(* Logix 5000 Program export BasicLaserCommands; software revision 21.03 *)

TYPE GENERIC :
STRUCT
   cmd : GENERIC_CMD;
   res : LSTRING;
   error : DINT;
END_STRUCT
END_TYPE

TYPE SIMPLECMD :
STRUCT
   cmd : EMPTY_CMD;
   res : LSTRING;
   error : DINT;
END_STRUCT
END_TYPE

TYPE GETCOUNT :
STRUCT
   cmd : GETID_CMD;
   res : DINT;
   error : DINT;
END_STRUCT
END_TYPE

TYPE GETVARIABLES :
STRUCT
   cmd : GETID_CMD;
   res : LSTRING;
   error : DINT;
END_STRUCT
END_TYPE

TYPE SETPOSITIONOFFSET :
STRUCT
   cmd : SETPOSITIONOFFSET_CMD;
   error : DINT;
END_STRUCT
END_TYPE

TYPE SETDATA :
STRUCT
   cmd : SETDATA_CMD;
   error : DINT;
END_STRUCT
END_TYPE

TYPE LSTRING :   // string type
STRUCT
   LEN : DINT;
   DATA : SINT[400];
END_STRUCT
END_TYPE

TYPE SETENCODERDELAY_CMD :
STRUCT
   value : LSTRING;
   global : BOOL;
   send : BOOL;
END_STRUCT
END_TYPE

TYPE GETCOUNTERVALUE :
STRUCT
   cmd : GETID_CMD;
   res : LSTRING;
   error : DINT;
END_STRUCT
END_TYPE

TYPE BasicLaserCommands :
STRUCT
   BEGINTRANS : NORES_CMD;
   EXECTRANS : NORES_CMD;
   GETCOUNT : GETCOUNT;
   SETCOUNT : SETCOUNT;
   GETCOUNTERVALUE : GETCOUNTERVALUE;
   SETCOUNTERVALUE : SETCOUNTERVALUE;
   GETPARSEDTEXT : GETPARSEDTEXT;
   GETTEXT : GETTEXT;
   SETTEXT : SETTEXT;
   GETVARLIST : SIMPLECMD;
   GETVARIABLES : GETVARIABLES;
   SETVARIABLES : SETVARIABLES;
   LOADPROJECT : LOADPROJECT;
   GETCURRENTPROJECT : SIMPLECMD;
   SAVEPROJECT : SAVEPROJECT;
   GETPOSITIONOFFSET : GETPOSITIONOFFSET;
   SETPOSITIONOFFSET : SETPOSITIONOFFSET;
   GETENCODERDELAY : GETENCODERDELAY;
   SETENCODERDELAY : SETENCODERDELAY;
   RESETSYSTEM : NORES_CMD;
   GETDATA : GETDATA;
   SETDATA : SETDATA;
   GETVERSION : GETVERSION;
   GENERIC : GENERIC;
   priv : LASER_PRIVATE_FIELDS;
END_STRUCT
END_TYPE

TYPE SAVEPROJECT :
STRUCT
   cmd : LOADPROJECT_CMD;
   error : DINT;
END_STRUCT
END_TYPE

TYPE LASER_PRIVATE_FIELDS :
STRUCT
   data : SINT[808];
   busy : BOOL;
END_STRUCT
END_TYPE

TYPE GETDATA_CMD :
STRUCT
   object : LSTRING;
   id : LSTRING;
   send : BOOL;
END_STRUCT
END_TYPE

TYPE GETENCODERDELAY :
STRUCT
   cmd : GETENCODERDELAY_CMD;
   res : LSTRING;
   error : DINT;
END_STRUCT
END_TYPE

TYPE SETCOUNT :
STRUCT
   cmd : SETCOUNT_CMD;
   error : DINT;
END_STRUCT
END_TYPE

TYPE GETID_CMD :
STRUCT
   ID : LSTRING;
   send : BOOL;
END_STRUCT
END_TYPE

TYPE POSITION :
STRUCT
   x : REAL;
   y : REAL;
END_STRUCT
END_TYPE

TYPE GETENCODERDELAY_CMD :
STRUCT
   global : BOOL;
   send : BOOL;
END_STRUCT
END_TYPE

TYPE SETDATA_CMD :
STRUCT
   object : LSTRING;
   id : LSTRING;
   data : LSTRING;
   send : BOOL;
END_STRUCT
END_TYPE

TYPE SETVARIABLES :
STRUCT
   cmd : SETID_CMD;
   error : DINT;
END_STRUCT
END_TYPE

TYPE GETDATA :
STRUCT
   cmd : GETDATA_CMD;
   res : LSTRING;
   error : DINT;
END_STRUCT
END_TYPE

TYPE GETPOSITIONOFFSET :
STRUCT
   cmd : EMPTY_CMD;
   res : POSITION;
   error : DINT;
END_STRUCT
END_TYPE

TYPE SETCOUNTERVALUE :
STRUCT
   cmd : SETID_CMD;
   error : DINT;
END_STRUCT
END_TYPE

TYPE SETPOSITIONOFFSET_CMD :
STRUCT
   pos : POSITION;
   send : BOOL;
END_STRUCT
END_TYPE

TYPE EMPTY_CMD :
STRUCT
   send : BOOL;
END_STRUCT
END_TYPE

TYPE SETENCODERDELAY :
STRUCT
   cmd : SETENCODERDELAY_CMD;
   error : DINT;
END_STRUCT
END_TYPE

TYPE SETID_CMD :
STRUCT
   ID : LSTRING;
   value : LSTRING;
   send : BOOL;
END_STRUCT
END_TYPE

TYPE LOADPROJECT :
STRUCT
   cmd : LOADPROJECT_CMD;
   error : DINT;
END_STRUCT
END_TYPE

TYPE LOADPROJECT_CMD :
STRUCT
   URI : LSTRING;
   send : BOOL;
END_STRUCT
END_TYPE

TYPE GETVERSION :
STRUCT
   cmd : EMPTY_CMD;
   res : GETVERSION_RES;
   error : DINT;
END_STRUCT
END_TYPE

TYPE SETTEXT_CMD :
STRUCT
   name : LSTRING;
   value : LSTRING;
   send : BOOL;
END_STRUCT
END_TYPE

TYPE GETVERSION_RES :
STRUCT
   software : LSTRING;
   dsp : LSTRING;
   image : LSTRING;
END_STRUCT
END_TYPE

TYPE GENERIC_CMD :
STRUCT
   command : LSTRING;
   arg2 : LSTRING;
   arg3 : LSTRING;
   arg4 : LSTRING;
   arg5 : LSTRING;
   send : BOOL;
END_STRUCT
END_TYPE

TYPE GETTEXT_CMD :
STRUCT
   name : LSTRING;
   send : BOOL;
END_STRUCT
END_TYPE

TYPE GETPARSEDTEXT :
STRUCT
   cmd : GETTEXT_CMD;
   res : LSTRING;
   error : DINT;
END_STRUCT
END_TYPE

TYPE SETTEXT :
STRUCT
   cmd : SETTEXT_CMD;
   error : DINT;
END_STRUCT
END_TYPE

TYPE SETCOUNT_CMD :
STRUCT
   ID : LSTRING;
   value : DINT;
   send : BOOL;
END_STRUCT
END_TYPE

TYPE NORES_CMD :
STRUCT
   cmd : EMPTY_CMD;
   error : DINT;
END_STRUCT
END_TYPE

TYPE GETTEXT :
STRUCT
   cmd : GETTEXT_CMD;
   res : LSTRING;
   error : DINT;
END_STRUCT
END_TYPE

ADD_ON_INSTRUCTION StrToArr   (* revision 1.0, vendor 1 *)
VAR_IN_OUT
   out : SINT[404]; {required}
   str : LSTRING; {required}
END_VAR
VAR_OUTPUT
   size : DINT; {access Read Only, required}
END_VAR

ROUTINE Logic   (* ladder *)
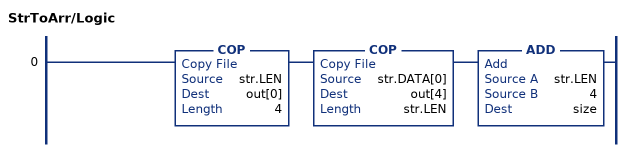
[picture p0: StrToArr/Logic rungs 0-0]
   0: COP(str.LEN,out[0],4)COP(str.DATA[0],out[4],str.LEN)ADD(str.LEN,4,size);
END_ROUTINE
END_ADD_ON_INSTRUCTION

ADD_ON_INSTRUCTION AppendStrs   (* revision 1.0, vendor 1 *)
VAR_IN_OUT
   str1 : LSTRING; {required}
   str2 : LSTRING; {required}
   out : SINT[808]; {required}
END_VAR
VAR_OUTPUT
   size : DINT; {access Read Only, required}
END_VAR
VAR
   cpy : StrToArr; {access None}
   n : DINT; {access None}
   offset : DINT; {access None}
   buf : SINT[404]; {access None}
END_VAR

ROUTINE Logic   (* ladder *)
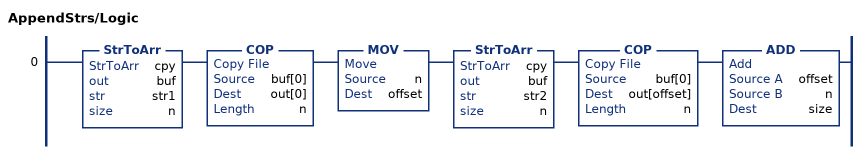
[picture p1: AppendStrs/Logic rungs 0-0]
   0: StrToArr(cpy,buf,str1,n)COP(buf[0],out[0],n)MOV(n,offset)StrToArr(cpy,buf,str2,n)COP(buf[0],out[offset],n)ADD(offset,n,size);
END_ROUTINE
END_ADD_ON_INSTRUCTION

ADD_ON_INSTRUCTION AppendStrs5   (* revision 1.0, vendor 1 *)
VAR_IN_OUT
   str1 : LSTRING; {required}
   str2 : LSTRING; {required}
   str3 : LSTRING; {required}
   str4 : LSTRING; {required}
   str5 : LSTRING; {required}
   out : SINT[808]; {required}
END_VAR
VAR_OUTPUT
   size : DINT; {access Read Only, required}
END_VAR
VAR_INPUT
   number_of_strings : DINT; {required}
   offset : DINT; {required}
END_VAR
VAR
   cpy : StrToArr; {access None}
   n : DINT; {access None}
   buf : SINT[404]; {access None}
END_VAR

ROUTINE Logic   (* ladder *)
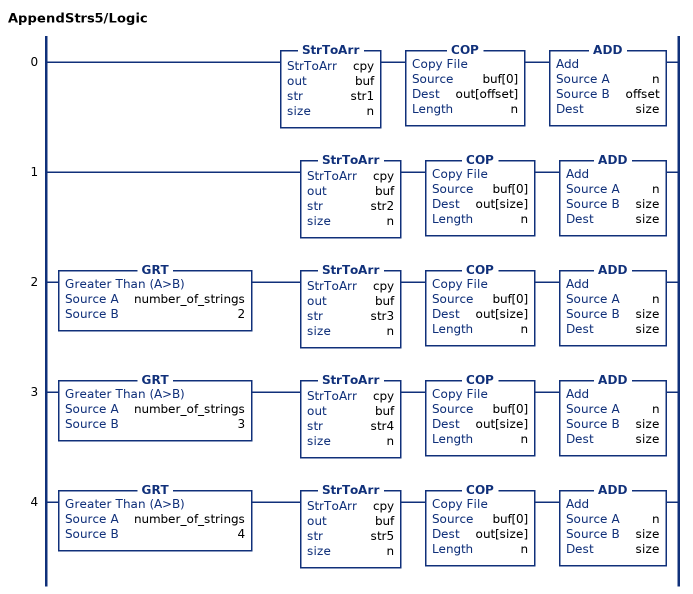
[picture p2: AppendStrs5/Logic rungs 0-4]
   0: StrToArr(cpy,buf,str1,n)COP(buf[0],out[offset],n)ADD(n,offset,size);
   1: StrToArr(cpy,buf,str2,n)COP(buf[0],out[size],n)ADD(n,size,size);
   2: GRT(number_of_strings,2)StrToArr(cpy,buf,str3,n)COP(buf[0],out[size],n)ADD(n,size,size);
   3: GRT(number_of_strings,3)StrToArr(cpy,buf,str4,n)COP(buf[0],out[size],n)ADD(n,size,size);
   4: GRT(number_of_strings,4)StrToArr(cpy,buf,str5,n)COP(buf[0],out[size],n)ADD(n,size,size);
END_ROUTINE
END_ADD_ON_INSTRUCTION

ADD_ON_INSTRUCTION ArrToStr   (* revision 1.0, vendor 1 *)
VAR_IN_OUT
   arr : SINT[404]; {required}
   out : LSTRING; {required}
END_VAR

ROUTINE Logic   (* ladder *)
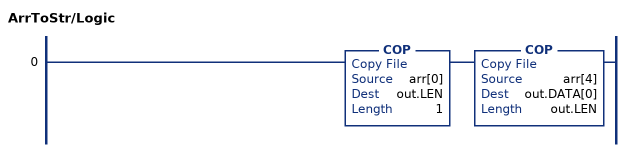
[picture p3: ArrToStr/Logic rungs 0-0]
   0: COP(arr[0],out.LEN,1)COP(arr[4],out.DATA[0],out.LEN);
END_ROUTINE
END_ADD_ON_INSTRUCTION

VAR_GLOBAL   (* controller tags *)
   Domino_internal_getvarlist : MESSAGE;
        MessageParameters(MessageType := CIP Generic, ConnectedFlag := 2, ConnectionPath := DFSeries, ServiceCode := 16#0054, ObjectType := 16#0064, TargetObject := 1, LocalElement := DFSeriesBasic.priv.data, DestinationTag := DFSeriesBasic.priv.data)
   Domino_internal_exectrans : MESSAGE;
        MessageParameters(MessageType := CIP Generic, ConnectedFlag := 2, ConnectionPath := DFSeries, ServiceCode := 16#004c, ObjectType := 16#0064, TargetObject := 1, LocalElement := DFSeriesBasic.priv, DestinationTag := DFSeriesBasic.priv)
   Domino_internal_gettext : MESSAGE;
        MessageParameters(MessageType := CIP Generic, RequestedLength := 101, ConnectedFlag := 2, ConnectionPath := DFSeries, ServiceCode := 16#0052, ObjectType := 16#0064, TargetObject := 1, LocalElement := DFSeriesBasic.priv, DestinationTag := DFSeriesBasic.priv)
   Domino_internal_loadproject : MESSAGE;
        MessageParameters(MessageType := CIP Generic, RequestedLength := 1, ConnectedFlag := 2, ConnectionPath := DFSeries, ServiceCode := 16#0057, ObjectType := 16#0064, TargetObject := 1, LocalElement := DFSeriesBasic.priv, DestinationTag := DFSeriesBasic.priv)
   Domino_internal_getcurrentproject : MESSAGE;
        MessageParameters(MessageType := CIP Generic, ConnectedFlag := 2, ConnectionPath := DFSeries, ServiceCode := 16#0058, ObjectType := 16#0064, TargetObject := 1, LocalElement := DFSeriesBasic.priv, DestinationTag := DFSeriesBasic.priv)
   Domino_internal_getpositionoffset : MESSAGE;
        MessageParameters(MessageType := CIP Generic, ConnectedFlag := 2, ConnectionPath := DFSeries, ServiceCode := 16#005a, ObjectType := 16#0064, TargetObject := 1, LocalElement := DFSeriesBasic.priv, DestinationTag := DFSeriesBasic.priv)
   Domino_internal_setcountervalue : MESSAGE;
        MessageParameters(MessageType := CIP Generic, RequestedLength := 1, ConnectedFlag := 2, ConnectionPath := DFSeries, ServiceCode := 16#0050, ObjectType := 16#0064, TargetObject := 1, LocalElement := DFSeriesBasic.priv, DestinationTag := DFSeriesBasic.priv)
   Domino_internal_setcount : MESSAGE;
        MessageParameters(MessageType := CIP Generic, RequestedLength := 1, ConnectedFlag := 2, ConnectionPath := DFSeries, ServiceCode := 16#004e, ObjectType := 16#0064, TargetObject := 1, LocalElement := DFSeriesBasic.priv, DestinationTag := DFSeriesBasic.priv)
   DFSeriesBasic : BasicLaserCommands;
   Domino_internal_resetsystem : MESSAGE;
        MessageParameters(MessageType := CIP Generic, ConnectedFlag := 2, ConnectionPath := DFSeries, ServiceCode := 16#005e, ObjectType := 16#0064, TargetObject := 1, LocalElement := DFSeriesBasic.priv, DestinationTag := DFSeriesBasic.priv)
   Domino_internal_getdata : MESSAGE;
        MessageParameters(MessageType := CIP Generic, RequestedLength := 1, ConnectedFlag := 2, ConnectionPath := DFSeries, ServiceCode := 16#005f, ObjectType := 16#0064, TargetObject := 1, LocalElement := DFSeriesBasic.priv, DestinationTag := DFSeriesBasic.priv)
   Domino_internal_getencoderdelay : MESSAGE;
        MessageParameters(MessageType := CIP Generic, RequestedLength := 1, ConnectedFlag := 2, ConnectionPath := DFSeries, ServiceCode := 16#005c, ObjectType := 16#0064, TargetObject := 1, LocalElement := DFSeriesBasic.priv, DestinationTag := DFSeriesBasic.priv)
   Domino_internal_generic : MESSAGE;
        MessageParameters(MessageType := CIP Generic, RequestedLength := 1, ConnectedFlag := 2, ConnectionPath := DFSeries, ServiceCode := 16#0063, ObjectType := 16#0064, TargetObject := 1, LocalElement := DFSeriesBasic.priv, DestinationTag := DFSeriesBasic.priv)
   Domino_internal_setvariables : MESSAGE;
        MessageParameters(MessageType := CIP Generic, RequestedLength := 1, ConnectedFlag := 2, ConnectionPath := DFSeries, ServiceCode := 16#0056, ObjectType := 16#0064, TargetObject := 1, LocalElement := DFSeriesBasic.priv, DestinationTag := DFSeriesBasic.priv)
   Domino_internal_getcountervalue : MESSAGE;
        MessageParameters(MessageType := CIP Generic, RequestedLength := 1, ConnectedFlag := 2, ConnectionPath := DFSeries, ServiceCode := 16#004f, ObjectType := 16#0064, TargetObject := 1, LocalElement := DFSeriesBasic.priv, DestinationTag := DFSeriesBasic.priv)
   Domino_internal_setpositionoffset : MESSAGE;
        MessageParameters(MessageType := CIP Generic, RequestedLength := 8, ConnectedFlag := 2, ConnectionPath := DFSeries, ServiceCode := 16#005b, ObjectType := 16#0064, TargetObject := 1, LocalElement := DFSeriesBasic.priv, DestinationTag := DFSeriesBasic.priv)
   Domino_internal_setencoderdelay : MESSAGE;
        MessageParameters(MessageType := CIP Generic, RequestedLength := 1, ConnectedFlag := 2, ConnectionPath := DFSeries, ServiceCode := 16#005d, ObjectType := 16#0064, TargetObject := 1, LocalElement := DFSeriesBasic.priv, DestinationTag := DFSeriesBasic.priv)
   Domino_internal_setdata : MESSAGE;
        MessageParameters(MessageType := CIP Generic, RequestedLength := 1, ConnectedFlag := 2, ConnectionPath := DFSeries, ServiceCode := 16#0060, ObjectType := 16#0064, TargetObject := 1, LocalElement := DFSeriesBasic.priv, DestinationTag := DFSeriesBasic.priv)
   Domino_internal_getparsedtext : MESSAGE;
        MessageParameters(MessageType := CIP Generic, RequestedLength := 1, ConnectedFlag := 2, ConnectionPath := DFSeries, ServiceCode := 16#0051, ObjectType := 16#0064, TargetObject := 1, LocalElement := DFSeriesBasic.priv, DestinationTag := DFSeriesBasic.priv)
   Domino_internal_getversion : MESSAGE;
        MessageParameters(MessageType := CIP Generic, ConnectedFlag := 2, ConnectionPath := DFSeries, ServiceCode := 16#0061, ObjectType := 16#0064, TargetObject := 1, LocalElement := DFSeriesBasic.priv, DestinationTag := DFSeriesBasic.priv)
   Domino_internal_begintrans : MESSAGE;
        MessageParameters(MessageType := CIP Generic, ConnectedFlag := 2, ConnectionPath := DFSeries, ServiceCode := 16#004b, ObjectType := 16#0064, TargetObject := 1, LocalElement := DFSeriesBasic.priv, DestinationTag := DFSeriesBasic.priv)
   Domino_internal_getvariables : MESSAGE;
        MessageParameters(MessageType := CIP Generic, RequestedLength := 1, ConnectedFlag := 2, ConnectionPath := DFSeries, ServiceCode := 16#0055, ObjectType := 16#0064, TargetObject := 1, LocalElement := DFSeriesBasic.priv, DestinationTag := DFSeriesBasic.priv)
   Domino_internal_settext : MESSAGE;
        MessageParameters(MessageType := CIP Generic, RequestedLength := 202, ConnectedFlag := 2, ConnectionPath := DFSeries, ServiceCode := 16#0053, ObjectType := 16#0064, TargetObject := 1, LocalElement := DFSeriesBasic.priv, DestinationTag := DFSeriesBasic.priv)
   Domino_internal_saveproject : MESSAGE;
        MessageParameters(MessageType := CIP Generic, RequestedLength := 1, ConnectedFlag := 2, ConnectionPath := DFSeries, ServiceCode := 16#0059, ObjectType := 16#0064, TargetObject := 1, LocalElement := DFSeriesBasic.priv, DestinationTag := DFSeriesBasic.priv)
   Domino_internal_getcount : MESSAGE;
        MessageParameters(MessageType := CIP Generic, RequestedLength := 1, ConnectedFlag := 2, ConnectionPath := DFSeries, ServiceCode := 16#004d, ObjectType := 16#0064, TargetObject := 1, LocalElement := DFSeriesBasic.priv, DestinationTag := DFSeriesBasic.priv)
END_VAR

PROGRAM BasicLaserCommands   (* main routine Main *)
VAR
   app : AppendStrs;
   app5 : AppendStrs5 := (number_of_strings := 3);
   len : DINT;
   n : DINT;
   toArr : StrToArr;
   toStr : ArrToStr;
END_VAR

ROUTINE Main   (* ladder *)
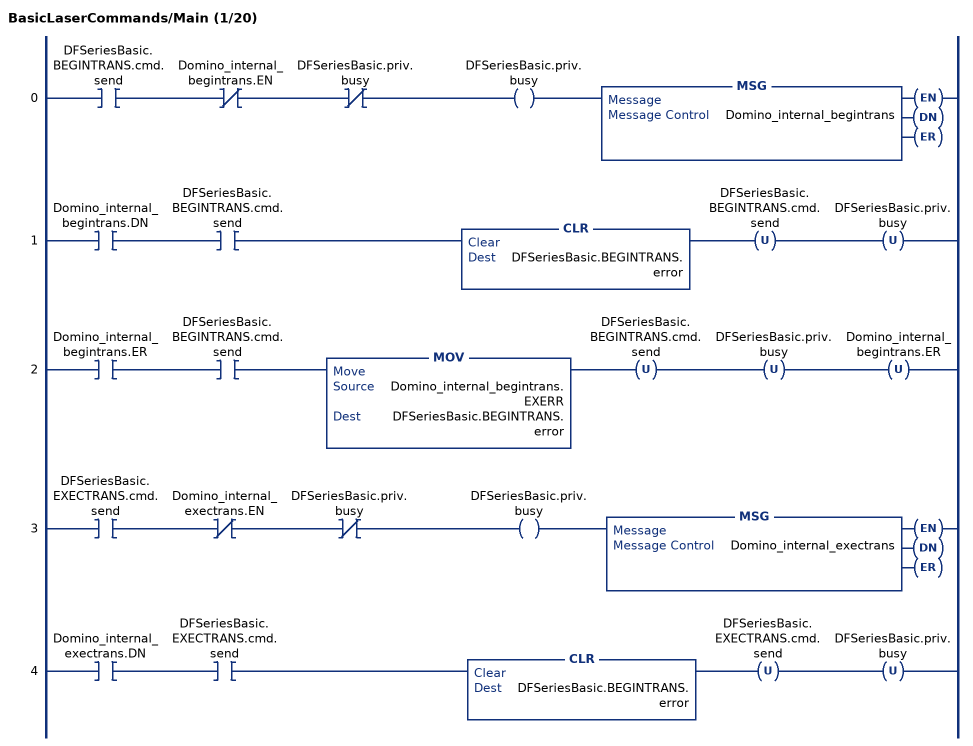
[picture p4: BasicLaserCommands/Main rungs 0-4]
   0: XIC(DFSeriesBasic.BEGINTRANS.cmd.send)XIO(Domino_internal_begintrans.EN)XIO(DFSeriesBasic.priv.busy)OTE(DFSeriesBasic.priv.busy)MSG(Domino_internal_begintrans);
   1: XIC(Domino_internal_begintrans.DN)XIC(DFSeriesBasic.BEGINTRANS.cmd.send)CLR(DFSeriesBasic.BEGINTRANS.error)OTU(DFSeriesBasic.BEGINTRANS.cmd.send)OTU(DFSeriesBasic.priv.busy);
   2: XIC(Domino_internal_begintrans.ER)XIC(DFSeriesBasic.BEGINTRANS.cmd.send)MOV(Domino_internal_begintrans.EXERR,DFSeriesBasic.BEGINTRANS.error)OTU(DFSeriesBasic.BEGINTRANS.cmd.send)OTU(DFSeriesBasic.priv.busy)OTU(Domino_internal_begintrans.ER);
   3: XIC(DFSeriesBasic.EXECTRANS.cmd.send)XIO(Domino_internal_exectrans.EN)XIO(DFSeriesBasic.priv.busy)OTE(DFSeriesBasic.priv.busy)MSG(Domino_internal_exectrans);
   4: XIC(Domino_internal_exectrans.DN)XIC(DFSeriesBasic.EXECTRANS.cmd.send)CLR(DFSeriesBasic.BEGINTRANS.error)OTU(DFSeriesBasic.EXECTRANS.cmd.send)OTU(DFSeriesBasic.priv.busy);
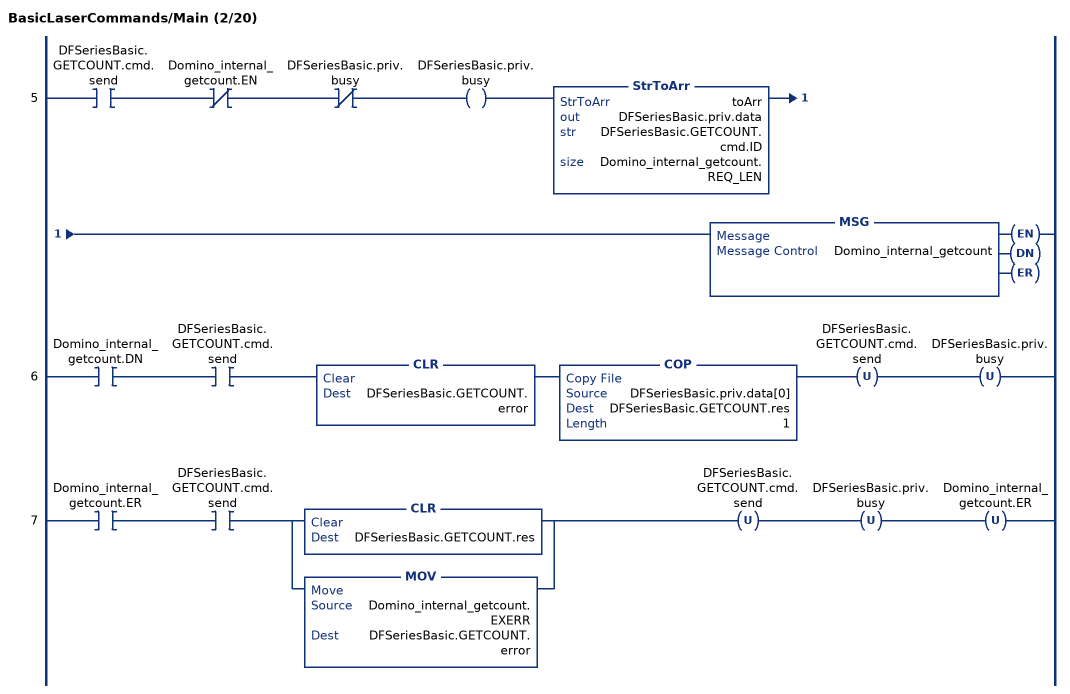
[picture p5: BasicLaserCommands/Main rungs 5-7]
   5: XIC(DFSeriesBasic.GETCOUNT.cmd.send)XIO(Domino_internal_getcount.EN)XIO(DFSeriesBasic.priv.busy)OTE(DFSeriesBasic.priv.busy)StrToArr(toArr,DFSeriesBasic.priv.data,DFSeriesBasic.GETCOUNT.cmd.ID,Domino_internal_getcount.REQ_LEN)MSG(Domino_internal_getcount);
   6: XIC(Domino_internal_getcount.DN)XIC(DFSeriesBasic.GETCOUNT.cmd.send)CLR(DFSeriesBasic.GETCOUNT.error)COP(DFSeriesBasic.priv.data[0],DFSeriesBasic.GETCOUNT.res,1)OTU(DFSeriesBasic.GETCOUNT.cmd.send)OTU(DFSeriesBasic.priv.busy);
   7: XIC(Domino_internal_getcount.ER)XIC(DFSeriesBasic.GETCOUNT.cmd.send)[CLR(DFSeriesBasic.GETCOUNT.res) ,MOV(Domino_internal_getcount.EXERR,DFSeriesBasic.GETCOUNT.error) ]OTU(DFSeriesBasic.GETCOUNT.cmd.send)OTU(DFSeriesBasic.priv.busy)OTU(Domino_internal_getcount.ER);
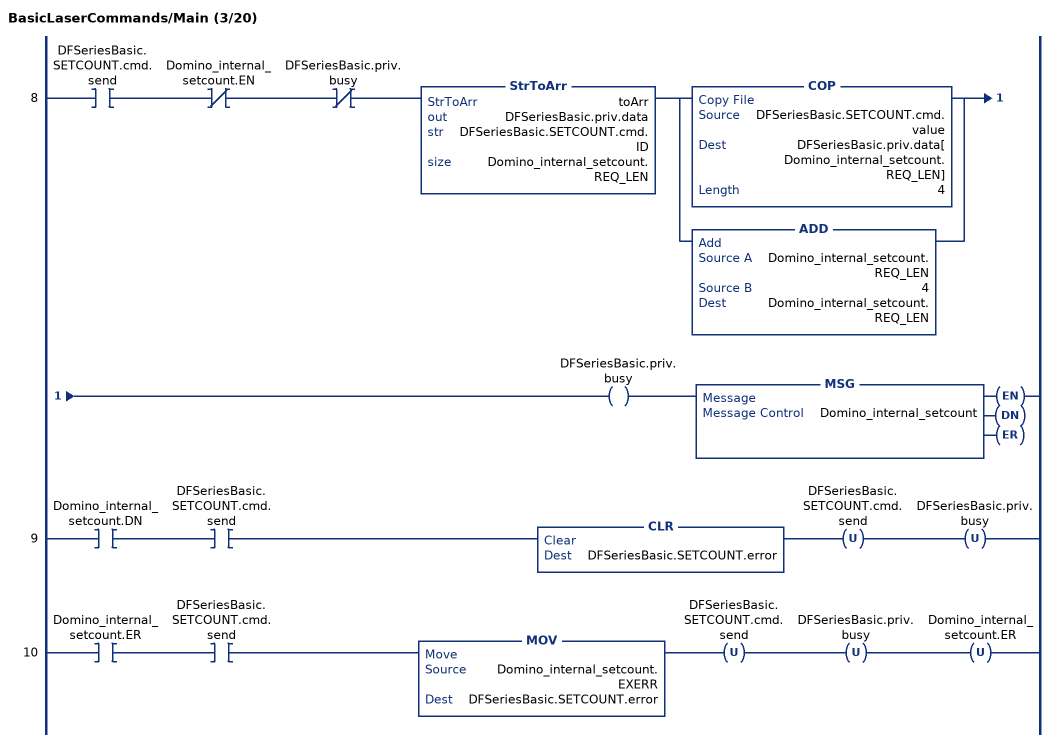
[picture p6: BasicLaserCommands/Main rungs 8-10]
   8: XIC(DFSeriesBasic.SETCOUNT.cmd.send)XIO(Domino_internal_setcount.EN)XIO(DFSeriesBasic.priv.busy)StrToArr(toArr,DFSeriesBasic.priv.data,DFSeriesBasic.SETCOUNT.cmd.ID,Domino_internal_setcount.REQ_LEN)[COP(DFSeriesBasic.SETCOUNT.cmd.value,DFSeriesBasic.priv.data[Domino_internal_setcount.REQ_LEN],4) ,ADD(Domino_internal_setcount.REQ_LEN,4,Domino_internal_setcount.REQ_LEN) ]OTE(DFSeriesBasic.priv.busy)MSG(Domino_internal_setcount);
   9: XIC(Domino_internal_setcount.DN)XIC(DFSeriesBasic.SETCOUNT.cmd.send)CLR(DFSeriesBasic.SETCOUNT.error)OTU(DFSeriesBasic.SETCOUNT.cmd.send)OTU(DFSeriesBasic.priv.busy);
   10: XIC(Domino_internal_setcount.ER)XIC(DFSeriesBasic.SETCOUNT.cmd.send)MOV(Domino_internal_setcount.EXERR,DFSeriesBasic.SETCOUNT.error)OTU(DFSeriesBasic.SETCOUNT.cmd.send)OTU(DFSeriesBasic.priv.busy)OTU(Domino_internal_setcount.ER);
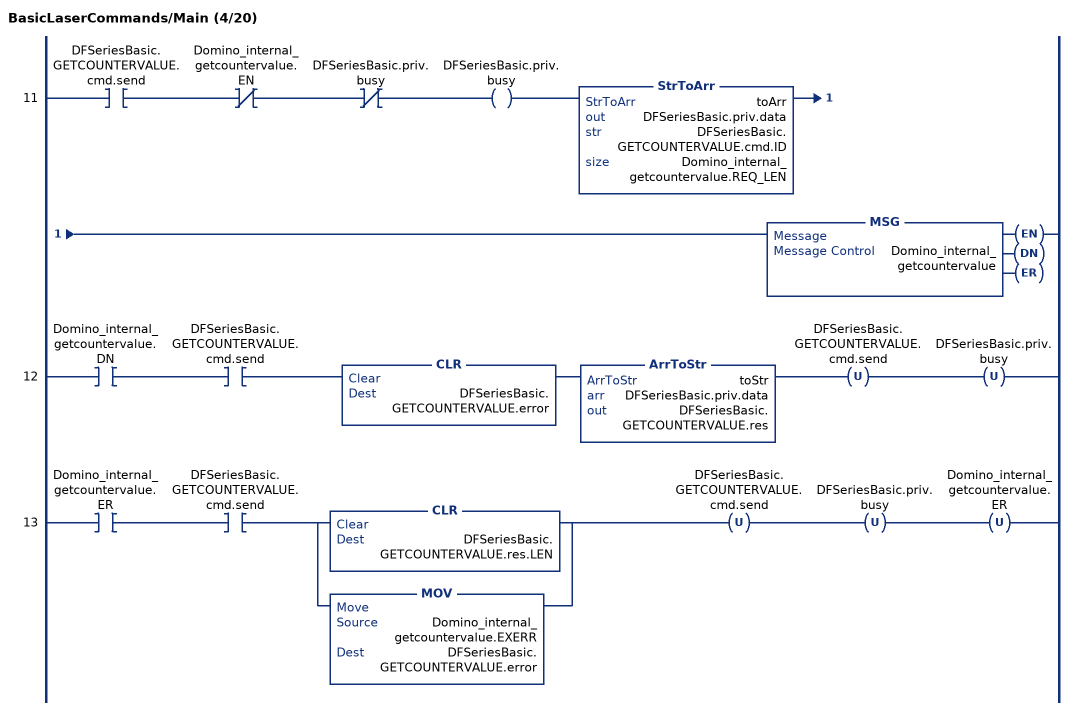
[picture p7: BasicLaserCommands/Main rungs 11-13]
   11: XIC(DFSeriesBasic.GETCOUNTERVALUE.cmd.send)XIO(Domino_internal_getcountervalue.EN)XIO(DFSeriesBasic.priv.busy)OTE(DFSeriesBasic.priv.busy)StrToArr(toArr,DFSeriesBasic.priv.data,DFSeriesBasic.GETCOUNTERVALUE.cmd.ID,Domino_internal_getcountervalue.REQ_LEN)MSG(Domino_internal_getcountervalue);
   12: XIC(Domino_internal_getcountervalue.DN)XIC(DFSeriesBasic.GETCOUNTERVALUE.cmd.send)CLR(DFSeriesBasic.GETCOUNTERVALUE.error)ArrToStr(toStr,DFSeriesBasic.priv.data,DFSeriesBasic.GETCOUNTERVALUE.res)OTU(DFSeriesBasic.GETCOUNTERVALUE.cmd.send)OTU(DFSeriesBasic.priv.busy);
   13: XIC(Domino_internal_getcountervalue.ER)XIC(DFSeriesBasic.GETCOUNTERVALUE.cmd.send)[CLR(DFSeriesBasic.GETCOUNTERVALUE.res.LEN) ,MOV(Domino_internal_getcountervalue.EXERR,DFSeriesBasic.GETCOUNTERVALUE.error) ]OTU(DFSeriesBasic.GETCOUNTERVALUE.cmd.send)OTU(DFSeriesBasic.priv.busy)OTU(Domino_internal_getcountervalue.ER);
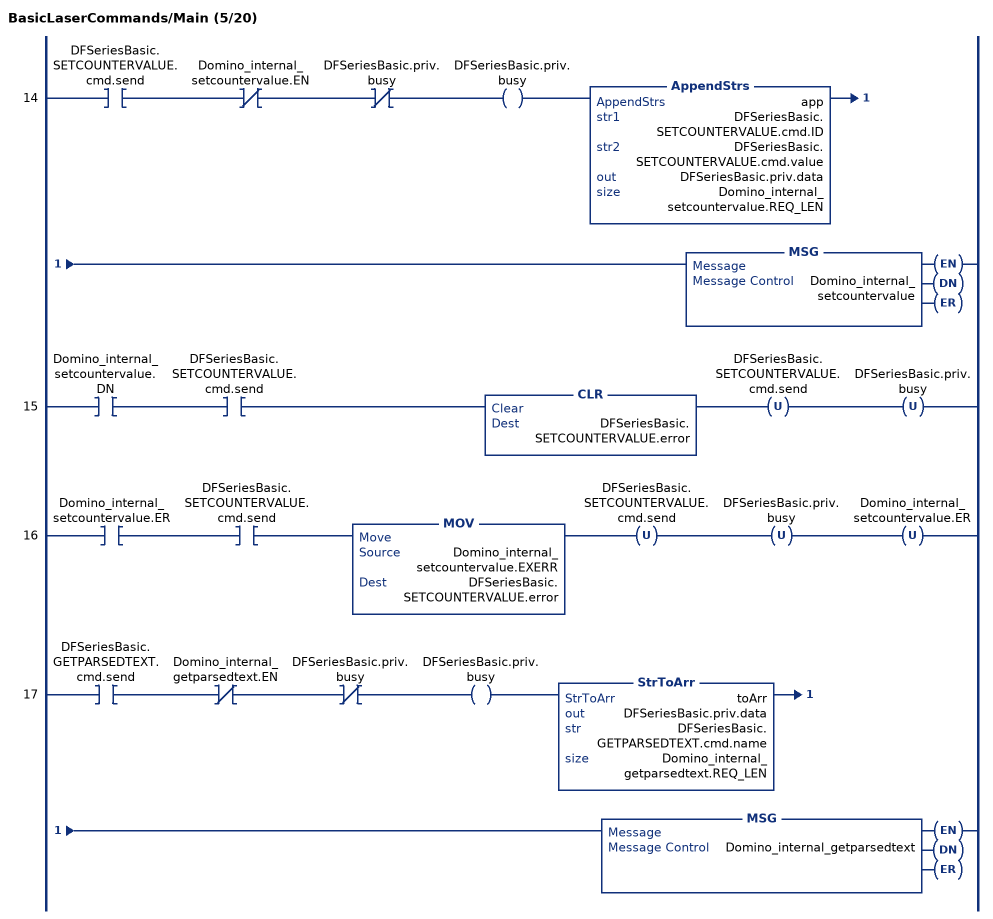
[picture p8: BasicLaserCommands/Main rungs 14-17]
   14: XIC(DFSeriesBasic.SETCOUNTERVALUE.cmd.send)XIO(Domino_internal_setcountervalue.EN)XIO(DFSeriesBasic.priv.busy)OTE(DFSeriesBasic.priv.busy)AppendStrs(app,DFSeriesBasic.SETCOUNTERVALUE.cmd.ID,DFSeriesBasic.SETCOUNTERVALUE.cmd.value,DFSeriesBasic.priv.data,Domino_internal_setcountervalue.REQ_LEN)MSG(Domino_internal_setcountervalue);
   15: XIC(Domino_internal_setcountervalue.DN)XIC(DFSeriesBasic.SETCOUNTERVALUE.cmd.send)CLR(DFSeriesBasic.SETCOUNTERVALUE.error)OTU(DFSeriesBasic.SETCOUNTERVALUE.cmd.send)OTU(DFSeriesBasic.priv.busy);
   16: XIC(Domino_internal_setcountervalue.ER)XIC(DFSeriesBasic.SETCOUNTERVALUE.cmd.send)MOV(Domino_internal_setcountervalue.EXERR,DFSeriesBasic.SETCOUNTERVALUE.error)OTU(DFSeriesBasic.SETCOUNTERVALUE.cmd.send)OTU(DFSeriesBasic.priv.busy)OTU(Domino_internal_setcountervalue.ER);
   17: XIC(DFSeriesBasic.GETPARSEDTEXT.cmd.send)XIO(Domino_internal_getparsedtext.EN)XIO(DFSeriesBasic.priv.busy)OTE(DFSeriesBasic.priv.busy)StrToArr(toArr,DFSeriesBasic.priv.data,DFSeriesBasic.GETPARSEDTEXT.cmd.name,Domino_internal_getparsedtext.REQ_LEN)MSG(Domino_internal_getparsedtext);
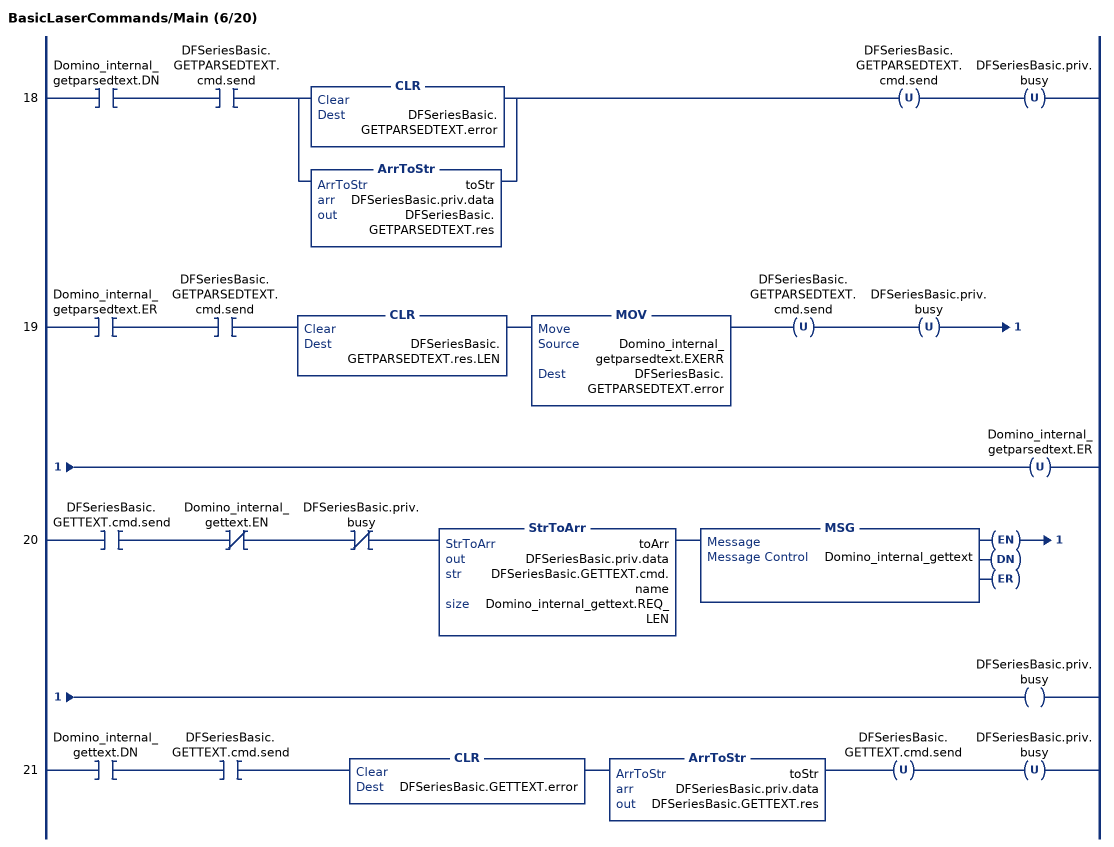
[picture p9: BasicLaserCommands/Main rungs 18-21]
   18: XIC(Domino_internal_getparsedtext.DN)XIC(DFSeriesBasic.GETPARSEDTEXT.cmd.send)[CLR(DFSeriesBasic.GETPARSEDTEXT.error) ,ArrToStr(toStr,DFSeriesBasic.priv.data,DFSeriesBasic.GETPARSEDTEXT.res) ]OTU(DFSeriesBasic.GETPARSEDTEXT.cmd.send)OTU(DFSeriesBasic.priv.busy);
   19: XIC(Domino_internal_getparsedtext.ER)XIC(DFSeriesBasic.GETPARSEDTEXT.cmd.send)CLR(DFSeriesBasic.GETPARSEDTEXT.res.LEN)MOV(Domino_internal_getparsedtext.EXERR,DFSeriesBasic.GETPARSEDTEXT.error)OTU(DFSeriesBasic.GETPARSEDTEXT.cmd.send)OTU(DFSeriesBasic.priv.busy)OTU(Domino_internal_getparsedtext.ER);
   20: XIC(DFSeriesBasic.GETTEXT.cmd.send)XIO(Domino_internal_gettext.EN)XIO(DFSeriesBasic.priv.busy)StrToArr(toArr,DFSeriesBasic.priv.data,DFSeriesBasic.GETTEXT.cmd.name,Domino_internal_gettext.REQ_LEN)MSG(Domino_internal_gettext)OTE(DFSeriesBasic.priv.busy);
   21: XIC(Domino_internal_gettext.DN)XIC(DFSeriesBasic.GETTEXT.cmd.send)CLR(DFSeriesBasic.GETTEXT.error)ArrToStr(toStr,DFSeriesBasic.priv.data,DFSeriesBasic.GETTEXT.res)OTU(DFSeriesBasic.GETTEXT.cmd.send)OTU(DFSeriesBasic.priv.busy);
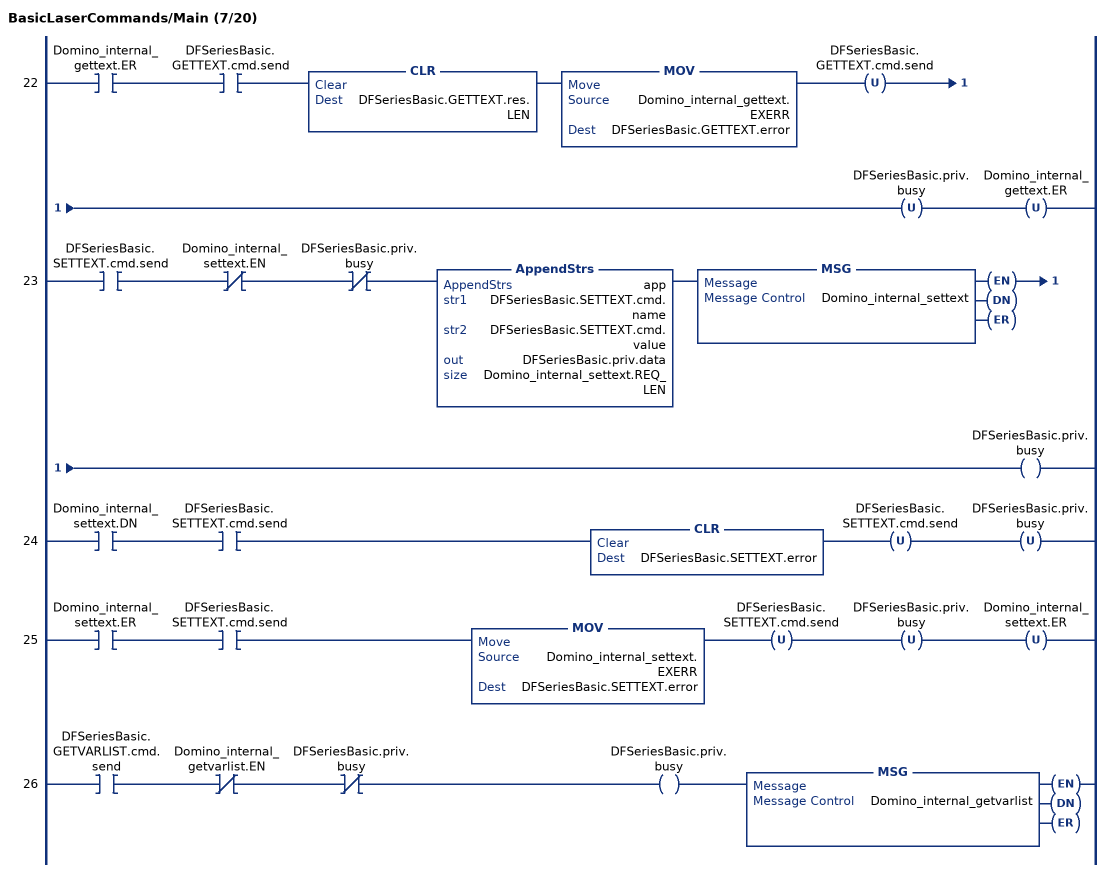
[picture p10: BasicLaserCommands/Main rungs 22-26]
   22: XIC(Domino_internal_gettext.ER)XIC(DFSeriesBasic.GETTEXT.cmd.send)CLR(DFSeriesBasic.GETTEXT.res.LEN)MOV(Domino_internal_gettext.EXERR,DFSeriesBasic.GETTEXT.error)OTU(DFSeriesBasic.GETTEXT.cmd.send)OTU(DFSeriesBasic.priv.busy)OTU(Domino_internal_gettext.ER);
   23: XIC(DFSeriesBasic.SETTEXT.cmd.send)XIO(Domino_internal_settext.EN)XIO(DFSeriesBasic.priv.busy)AppendStrs(app,DFSeriesBasic.SETTEXT.cmd.name,DFSeriesBasic.SETTEXT.cmd.value,DFSeriesBasic.priv.data,Domino_internal_settext.REQ_LEN)MSG(Domino_internal_settext)OTE(DFSeriesBasic.priv.busy);
   24: XIC(Domino_internal_settext.DN)XIC(DFSeriesBasic.SETTEXT.cmd.send)CLR(DFSeriesBasic.SETTEXT.error)OTU(DFSeriesBasic.SETTEXT.cmd.send)OTU(DFSeriesBasic.priv.busy);
   25: XIC(Domino_internal_settext.ER)XIC(DFSeriesBasic.SETTEXT.cmd.send)MOV(Domino_internal_settext.EXERR,DFSeriesBasic.SETTEXT.error)OTU(DFSeriesBasic.SETTEXT.cmd.send)OTU(DFSeriesBasic.priv.busy)OTU(Domino_internal_settext.ER);
   26: XIC(DFSeriesBasic.GETVARLIST.cmd.send)XIO(Domino_internal_getvarlist.EN)XIO(DFSeriesBasic.priv.busy)OTE(DFSeriesBasic.priv.busy)MSG(Domino_internal_getvarlist);
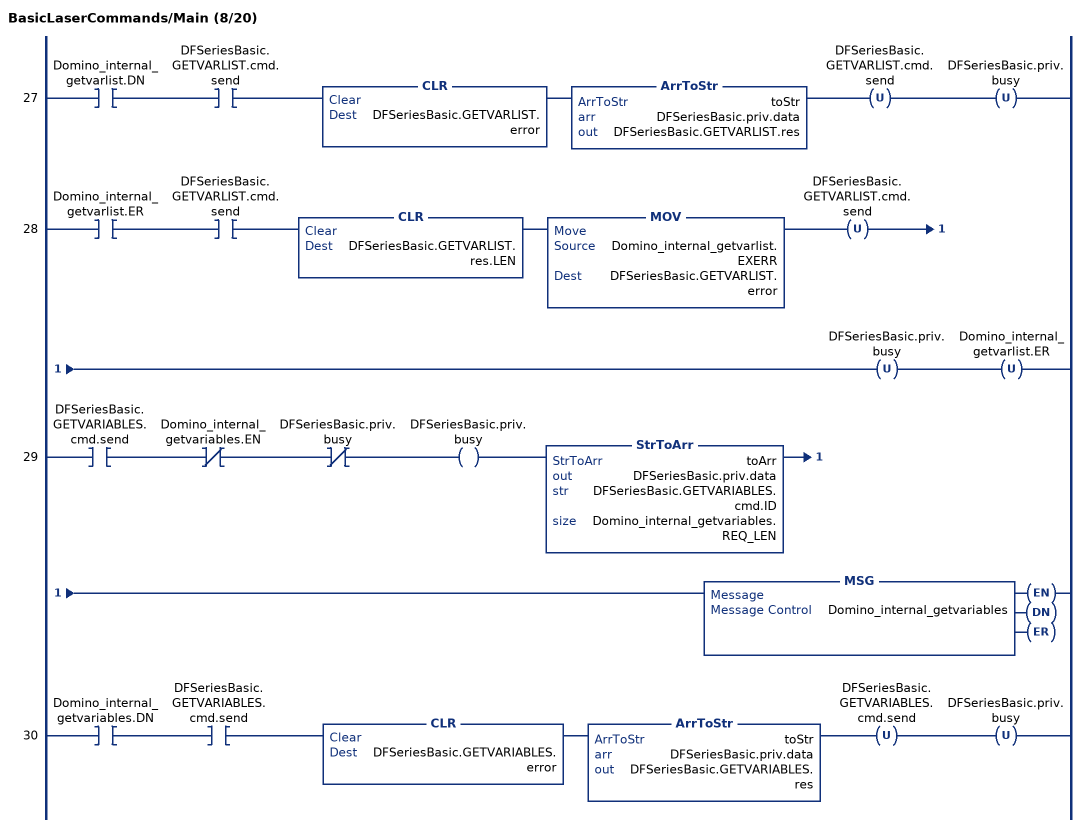
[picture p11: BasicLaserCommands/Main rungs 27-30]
   27: XIC(Domino_internal_getvarlist.DN)XIC(DFSeriesBasic.GETVARLIST.cmd.send)CLR(DFSeriesBasic.GETVARLIST.error)ArrToStr(toStr,DFSeriesBasic.priv.data,DFSeriesBasic.GETVARLIST.res)OTU(DFSeriesBasic.GETVARLIST.cmd.send)OTU(DFSeriesBasic.priv.busy);
   28: XIC(Domino_internal_getvarlist.ER)XIC(DFSeriesBasic.GETVARLIST.cmd.send)CLR(DFSeriesBasic.GETVARLIST.res.LEN)MOV(Domino_internal_getvarlist.EXERR,DFSeriesBasic.GETVARLIST.error)OTU(DFSeriesBasic.GETVARLIST.cmd.send)OTU(DFSeriesBasic.priv.busy)OTU(Domino_internal_getvarlist.ER);
   29: XIC(DFSeriesBasic.GETVARIABLES.cmd.send)XIO(Domino_internal_getvariables.EN)XIO(DFSeriesBasic.priv.busy)OTE(DFSeriesBasic.priv.busy)StrToArr(toArr,DFSeriesBasic.priv.data,DFSeriesBasic.GETVARIABLES.cmd.ID,Domino_internal_getvariables.REQ_LEN)MSG(Domino_internal_getvariables);
   30: XIC(Domino_internal_getvariables.DN)XIC(DFSeriesBasic.GETVARIABLES.cmd.send)CLR(DFSeriesBasic.GETVARIABLES.error)ArrToStr(toStr,DFSeriesBasic.priv.data,DFSeriesBasic.GETVARIABLES.res)OTU(DFSeriesBasic.GETVARIABLES.cmd.send)OTU(DFSeriesBasic.priv.busy);
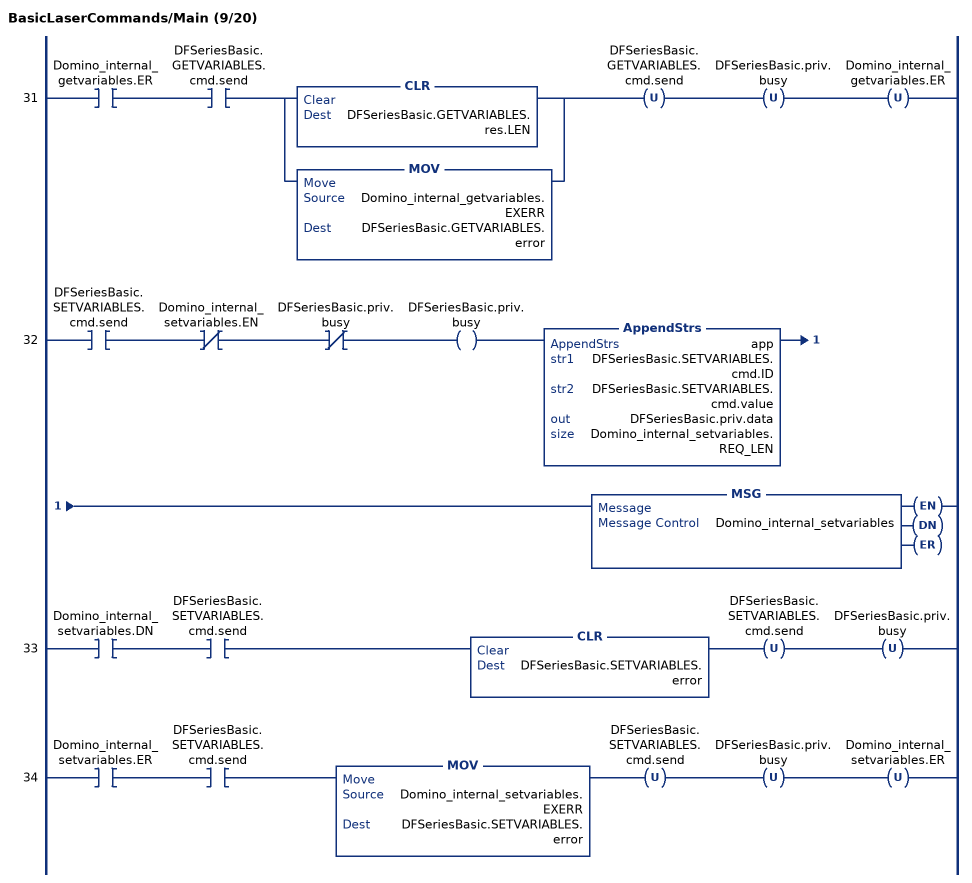
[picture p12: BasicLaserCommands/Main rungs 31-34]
   31: XIC(Domino_internal_getvariables.ER)XIC(DFSeriesBasic.GETVARIABLES.cmd.send)[CLR(DFSeriesBasic.GETVARIABLES.res.LEN) ,MOV(Domino_internal_getvariables.EXERR,DFSeriesBasic.GETVARIABLES.error) ]OTU(DFSeriesBasic.GETVARIABLES.cmd.send)OTU(DFSeriesBasic.priv.busy)OTU(Domino_internal_getvariables.ER);
   32: XIC(DFSeriesBasic.SETVARIABLES.cmd.send)XIO(Domino_internal_setvariables.EN)XIO(DFSeriesBasic.priv.busy)OTE(DFSeriesBasic.priv.busy)AppendStrs(app,DFSeriesBasic.SETVARIABLES.cmd.ID,DFSeriesBasic.SETVARIABLES.cmd.value,DFSeriesBasic.priv.data,Domino_internal_setvariables.REQ_LEN)MSG(Domino_internal_setvariables);
   33: XIC(Domino_internal_setvariables.DN)XIC(DFSeriesBasic.SETVARIABLES.cmd.send)CLR(DFSeriesBasic.SETVARIABLES.error)OTU(DFSeriesBasic.SETVARIABLES.cmd.send)OTU(DFSeriesBasic.priv.busy);
   34: XIC(Domino_internal_setvariables.ER)XIC(DFSeriesBasic.SETVARIABLES.cmd.send)MOV(Domino_internal_setvariables.EXERR,DFSeriesBasic.SETVARIABLES.error)OTU(DFSeriesBasic.SETVARIABLES.cmd.send)OTU(DFSeriesBasic.priv.busy)OTU(Domino_internal_setvariables.ER);
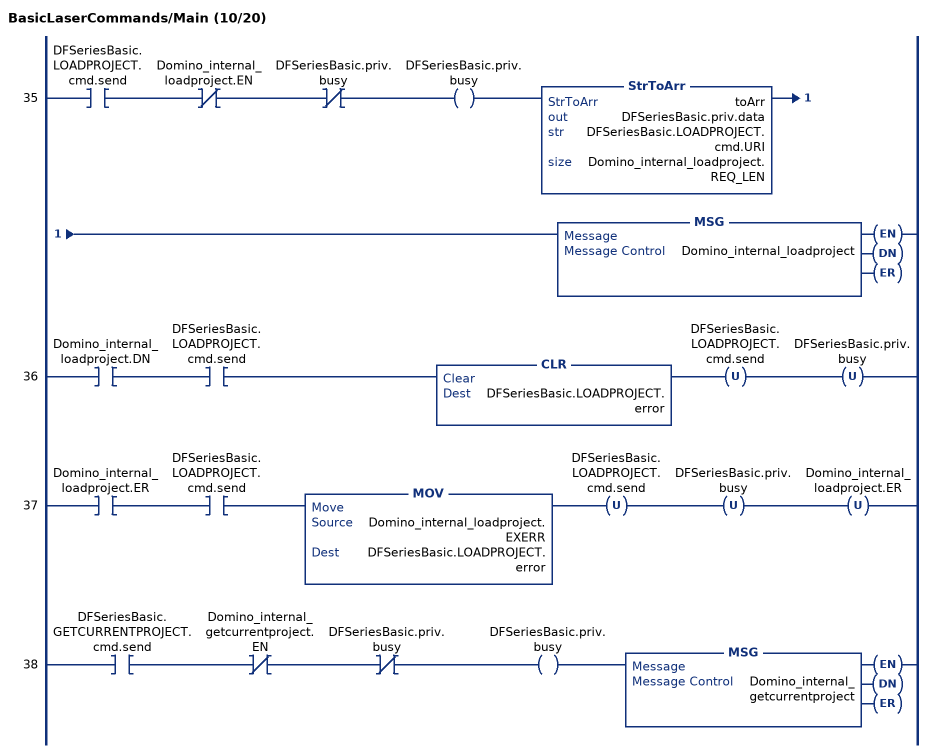
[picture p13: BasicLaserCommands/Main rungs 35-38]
   35: XIC(DFSeriesBasic.LOADPROJECT.cmd.send)XIO(Domino_internal_loadproject.EN)XIO(DFSeriesBasic.priv.busy)OTE(DFSeriesBasic.priv.busy)StrToArr(toArr,DFSeriesBasic.priv.data,DFSeriesBasic.LOADPROJECT.cmd.URI,Domino_internal_loadproject.REQ_LEN)MSG(Domino_internal_loadproject);
   36: XIC(Domino_internal_loadproject.DN)XIC(DFSeriesBasic.LOADPROJECT.cmd.send)CLR(DFSeriesBasic.LOADPROJECT.error)OTU(DFSeriesBasic.LOADPROJECT.cmd.send)OTU(DFSeriesBasic.priv.busy);
   37: XIC(Domino_internal_loadproject.ER)XIC(DFSeriesBasic.LOADPROJECT.cmd.send)MOV(Domino_internal_loadproject.EXERR,DFSeriesBasic.LOADPROJECT.error)OTU(DFSeriesBasic.LOADPROJECT.cmd.send)OTU(DFSeriesBasic.priv.busy)OTU(Domino_internal_loadproject.ER);
   38: XIC(DFSeriesBasic.GETCURRENTPROJECT.cmd.send)XIO(Domino_internal_getcurrentproject.EN)XIO(DFSeriesBasic.priv.busy)OTE(DFSeriesBasic.priv.busy)MSG(Domino_internal_getcurrentproject);
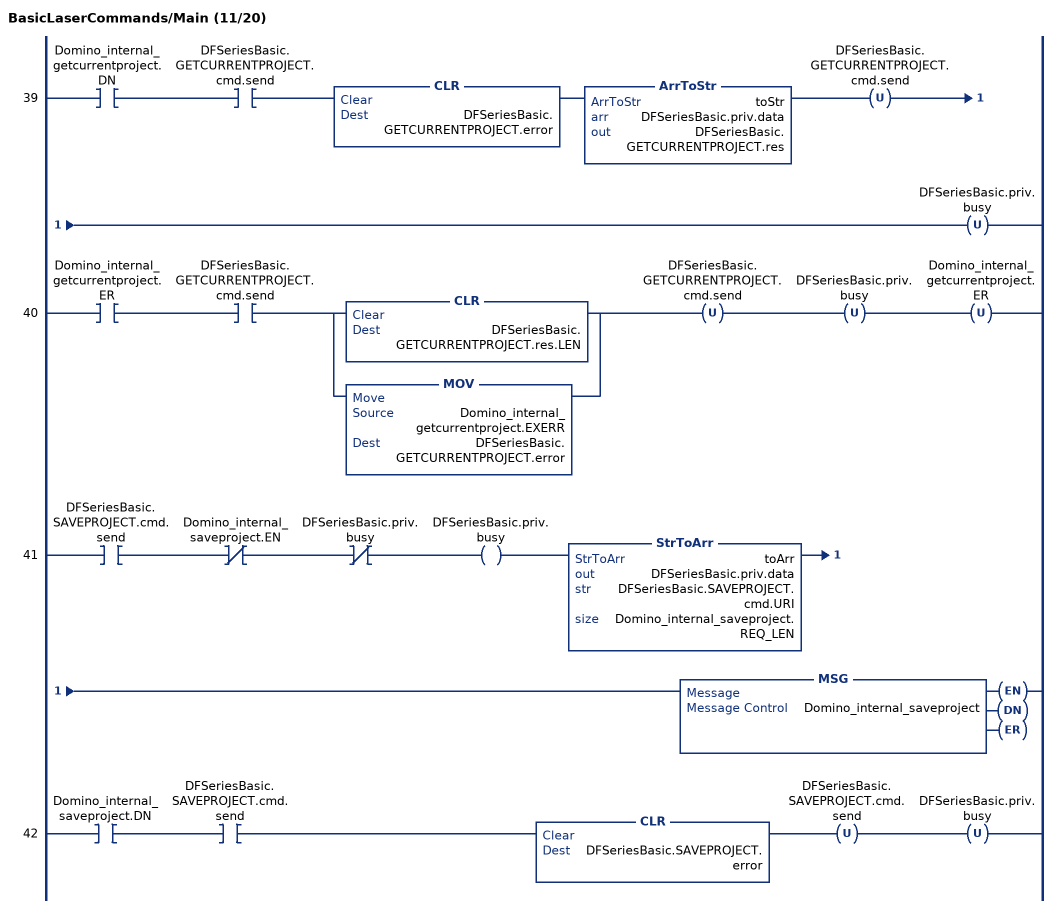
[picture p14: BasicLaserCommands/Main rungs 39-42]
   39: XIC(Domino_internal_getcurrentproject.DN)XIC(DFSeriesBasic.GETCURRENTPROJECT.cmd.send)CLR(DFSeriesBasic.GETCURRENTPROJECT.error)ArrToStr(toStr,DFSeriesBasic.priv.data,DFSeriesBasic.GETCURRENTPROJECT.res)OTU(DFSeriesBasic.GETCURRENTPROJECT.cmd.send)OTU(DFSeriesBasic.priv.busy);
   40: XIC(Domino_internal_getcurrentproject.ER)XIC(DFSeriesBasic.GETCURRENTPROJECT.cmd.send)[CLR(DFSeriesBasic.GETCURRENTPROJECT.res.LEN) ,MOV(Domino_internal_getcurrentproject.EXERR,DFSeriesBasic.GETCURRENTPROJECT.error) ]OTU(DFSeriesBasic.GETCURRENTPROJECT.cmd.send)OTU(DFSeriesBasic.priv.busy)OTU(Domino_internal_getcurrentproject.ER);
   41: XIC(DFSeriesBasic.SAVEPROJECT.cmd.send)XIO(Domino_internal_saveproject.EN)XIO(DFSeriesBasic.priv.busy)OTE(DFSeriesBasic.priv.busy)StrToArr(toArr,DFSeriesBasic.priv.data,DFSeriesBasic.SAVEPROJECT.cmd.URI,Domino_internal_saveproject.REQ_LEN)MSG(Domino_internal_saveproject);
   42: XIC(Domino_internal_saveproject.DN)XIC(DFSeriesBasic.SAVEPROJECT.cmd.send)CLR(DFSeriesBasic.SAVEPROJECT.error)OTU(DFSeriesBasic.SAVEPROJECT.cmd.send)OTU(DFSeriesBasic.priv.busy);
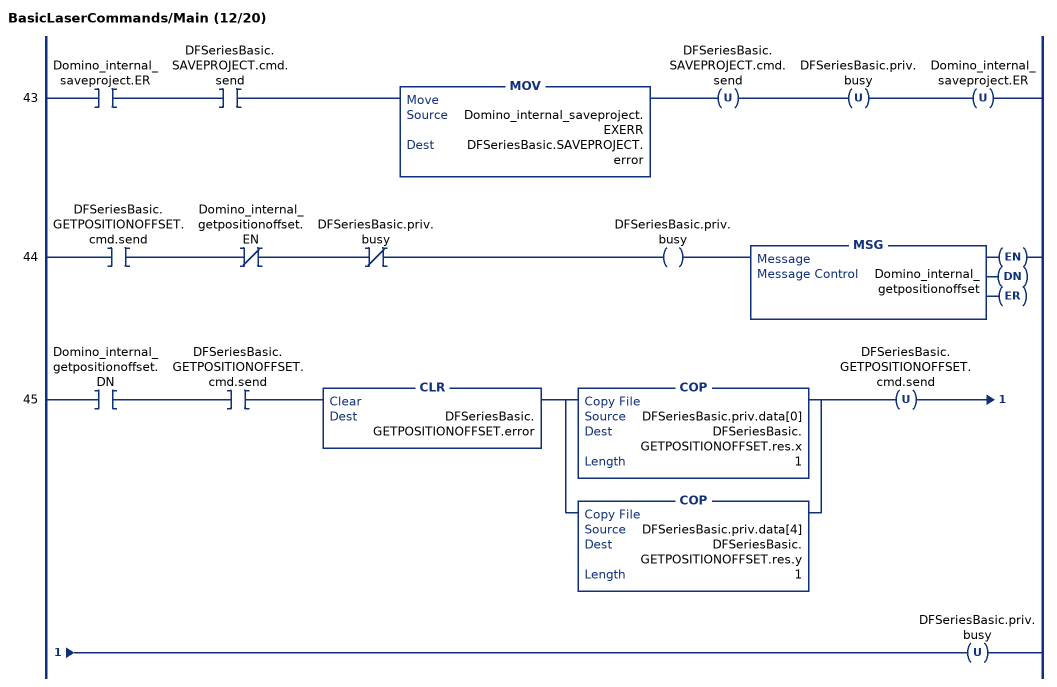
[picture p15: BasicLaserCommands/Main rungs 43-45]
   43: XIC(Domino_internal_saveproject.ER)XIC(DFSeriesBasic.SAVEPROJECT.cmd.send)MOV(Domino_internal_saveproject.EXERR,DFSeriesBasic.SAVEPROJECT.error)OTU(DFSeriesBasic.SAVEPROJECT.cmd.send)OTU(DFSeriesBasic.priv.busy)OTU(Domino_internal_saveproject.ER);
   44: XIC(DFSeriesBasic.GETPOSITIONOFFSET.cmd.send)XIO(Domino_internal_getpositionoffset.EN)XIO(DFSeriesBasic.priv.busy)OTE(DFSeriesBasic.priv.busy)MSG(Domino_internal_getpositionoffset);
   45: XIC(Domino_internal_getpositionoffset.DN)XIC(DFSeriesBasic.GETPOSITIONOFFSET.cmd.send)CLR(DFSeriesBasic.GETPOSITIONOFFSET.error)[COP(DFSeriesBasic.priv.data[0],DFSeriesBasic.GETPOSITIONOFFSET.res.x,1) ,COP(DFSeriesBasic.priv.data[4],DFSeriesBasic.GETPOSITIONOFFSET.res.y,1) ]OTU(DFSeriesBasic.GETPOSITIONOFFSET.cmd.send)OTU(DFSeriesBasic.priv.busy);
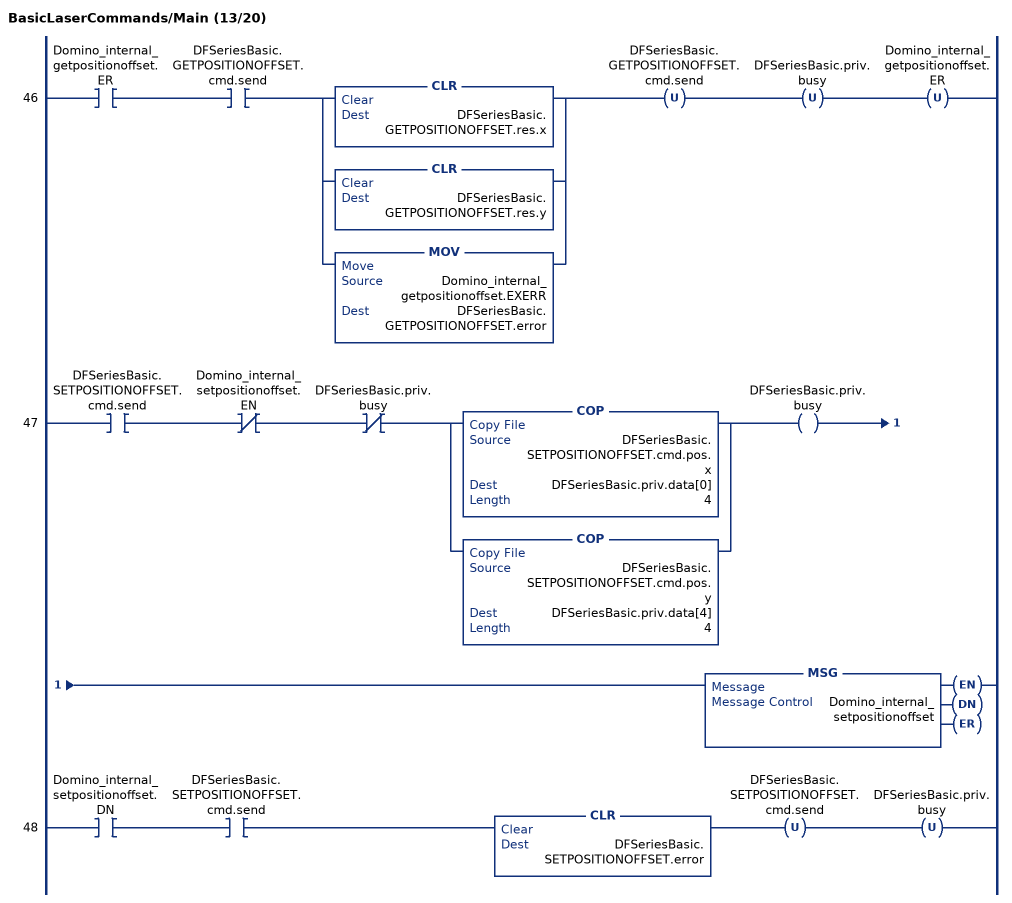
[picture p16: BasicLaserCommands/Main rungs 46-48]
   46: XIC(Domino_internal_getpositionoffset.ER)XIC(DFSeriesBasic.GETPOSITIONOFFSET.cmd.send)[CLR(DFSeriesBasic.GETPOSITIONOFFSET.res.x) ,CLR(DFSeriesBasic.GETPOSITIONOFFSET.res.y) ,MOV(Domino_internal_getpositionoffset.EXERR,DFSeriesBasic.GETPOSITIONOFFSET.error) ]OTU(DFSeriesBasic.GETPOSITIONOFFSET.cmd.send)OTU(DFSeriesBasic.priv.busy)OTU(Domino_internal_getpositionoffset.ER);
   47: XIC(DFSeriesBasic.SETPOSITIONOFFSET.cmd.send)XIO(Domino_internal_setpositionoffset.EN)XIO(DFSeriesBasic.priv.busy)[COP(DFSeriesBasic.SETPOSITIONOFFSET.cmd.pos.x,DFSeriesBasic.priv.data[0],4) ,COP(DFSeriesBasic.SETPOSITIONOFFSET.cmd.pos.y,DFSeriesBasic.priv.data[4],4) ]OTE(DFSeriesBasic.priv.busy)MSG(Domino_internal_setpositionoffset);
   48: XIC(Domino_internal_setpositionoffset.DN)XIC(DFSeriesBasic.SETPOSITIONOFFSET.cmd.send)CLR(DFSeriesBasic.SETPOSITIONOFFSET.error)OTU(DFSeriesBasic.SETPOSITIONOFFSET.cmd.send)OTU(DFSeriesBasic.priv.busy);
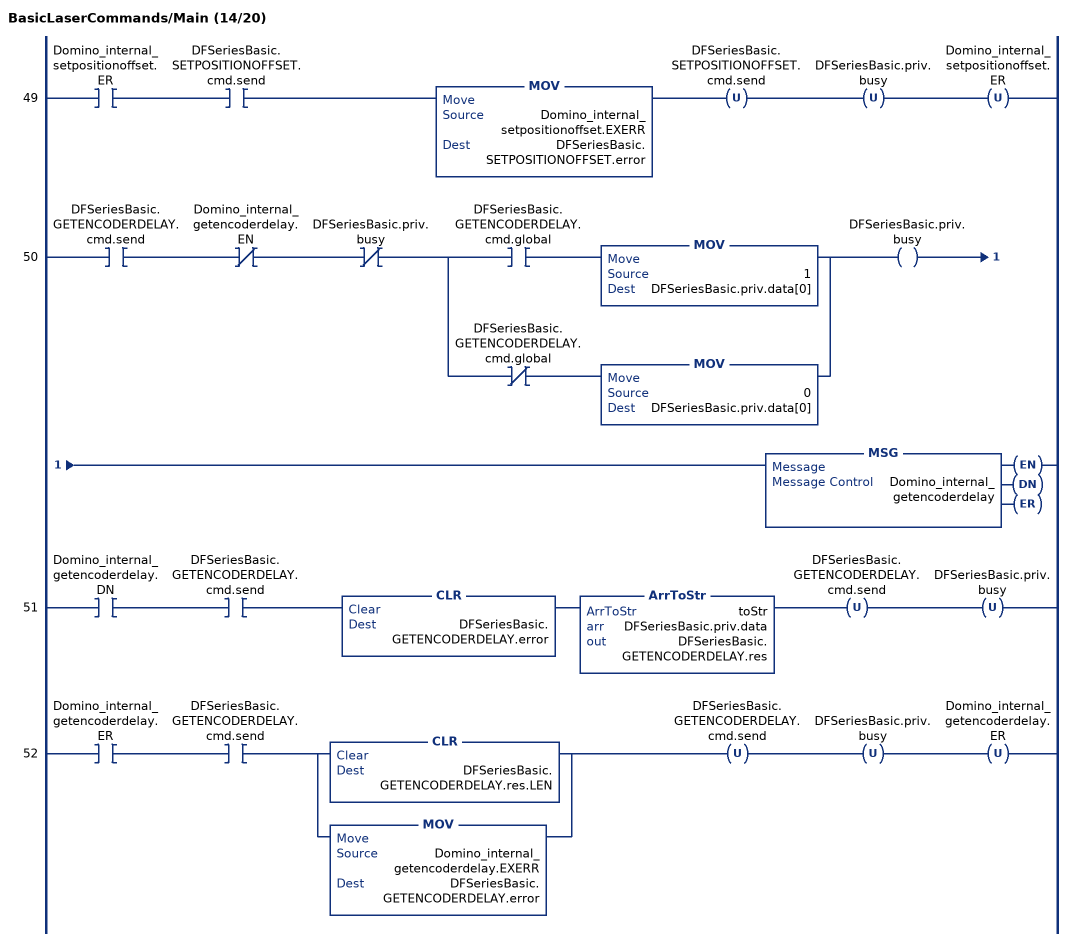
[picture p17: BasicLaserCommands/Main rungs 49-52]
   49: XIC(Domino_internal_setpositionoffset.ER)XIC(DFSeriesBasic.SETPOSITIONOFFSET.cmd.send)MOV(Domino_internal_setpositionoffset.EXERR,DFSeriesBasic.SETPOSITIONOFFSET.error)OTU(DFSeriesBasic.SETPOSITIONOFFSET.cmd.send)OTU(DFSeriesBasic.priv.busy)OTU(Domino_internal_setpositionoffset.ER);
   50: XIC(DFSeriesBasic.GETENCODERDELAY.cmd.send)XIO(Domino_internal_getencoderdelay.EN)XIO(DFSeriesBasic.priv.busy)[XIC(DFSeriesBasic.GETENCODERDELAY.cmd.global) MOV(1,DFSeriesBasic.priv.data[0]) ,XIO(DFSeriesBasic.GETENCODERDELAY.cmd.global) MOV(0,DFSeriesBasic.priv.data[0]) ]OTE(DFSeriesBasic.priv.busy)MSG(Domino_internal_getencoderdelay);
   51: XIC(Domino_internal_getencoderdelay.DN)XIC(DFSeriesBasic.GETENCODERDELAY.cmd.send)CLR(DFSeriesBasic.GETENCODERDELAY.error)ArrToStr(toStr,DFSeriesBasic.priv.data,DFSeriesBasic.GETENCODERDELAY.res)OTU(DFSeriesBasic.GETENCODERDELAY.cmd.send)OTU(DFSeriesBasic.priv.busy);
   52: XIC(Domino_internal_getencoderdelay.ER)XIC(DFSeriesBasic.GETENCODERDELAY.cmd.send)[CLR(DFSeriesBasic.GETENCODERDELAY.res.LEN) ,MOV(Domino_internal_getencoderdelay.EXERR,DFSeriesBasic.GETENCODERDELAY.error) ]OTU(DFSeriesBasic.GETENCODERDELAY.cmd.send)OTU(DFSeriesBasic.priv.busy)OTU(Domino_internal_getencoderdelay.ER);
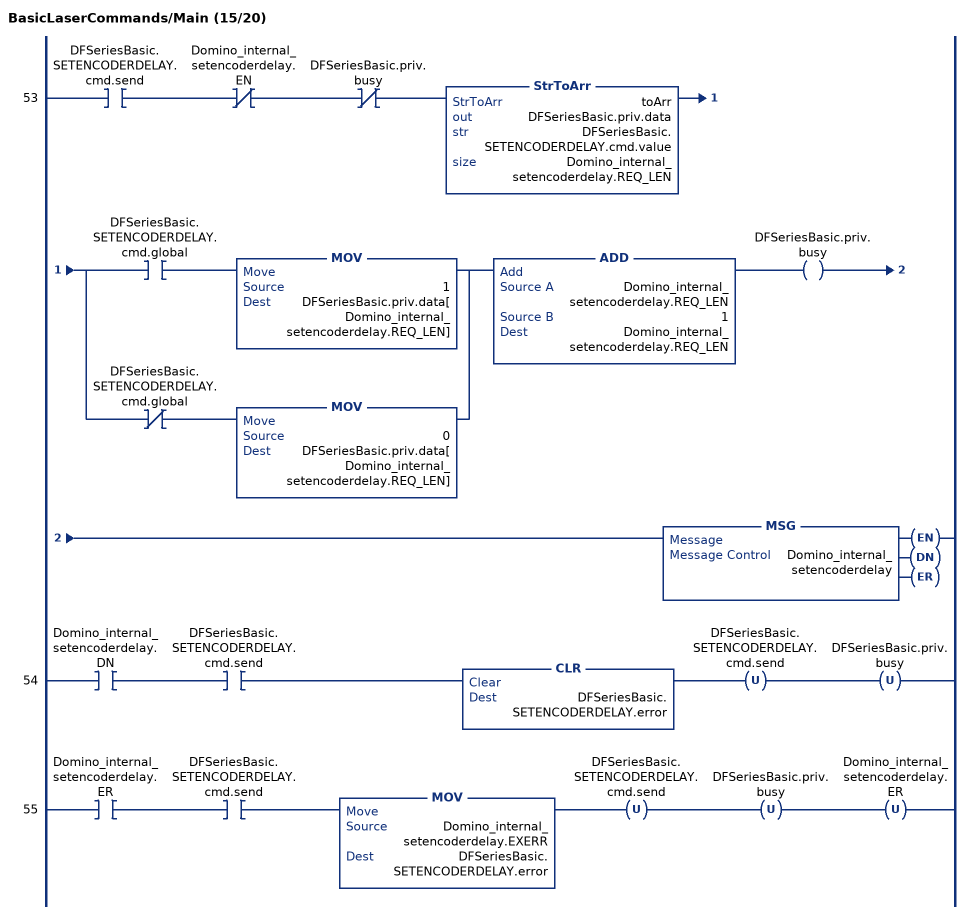
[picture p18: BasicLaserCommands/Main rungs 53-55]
   53: XIC(DFSeriesBasic.SETENCODERDELAY.cmd.send)XIO(Domino_internal_setencoderdelay.EN)XIO(DFSeriesBasic.priv.busy)StrToArr(toArr,DFSeriesBasic.priv.data,DFSeriesBasic.SETENCODERDELAY.cmd.value,Domino_internal_setencoderdelay.REQ_LEN)[XIC(DFSeriesBasic.SETENCODERDELAY.cmd.global) MOV(1,DFSeriesBasic.priv.data[Domino_internal_setencoderdelay.REQ_LEN]) ,XIO(DFSeriesBasic.SETENCODERDELAY.cmd.global) MOV(0,DFSeriesBasic.priv.data[Domino_internal_setencoderdelay.REQ_LEN]) ]ADD(Domino_internal_setencoderdelay.REQ_LEN,1,Domino_internal_setencoderdelay.REQ_LEN)OTE(DFSeriesBasic.priv.busy)MSG(Domino_internal_setencoderdelay);
   54: XIC(Domino_internal_setencoderdelay.DN)XIC(DFSeriesBasic.SETENCODERDELAY.cmd.send)CLR(DFSeriesBasic.SETENCODERDELAY.error)OTU(DFSeriesBasic.SETENCODERDELAY.cmd.send)OTU(DFSeriesBasic.priv.busy);
   55: XIC(Domino_internal_setencoderdelay.ER)XIC(DFSeriesBasic.SETENCODERDELAY.cmd.send)MOV(Domino_internal_setencoderdelay.EXERR,DFSeriesBasic.SETENCODERDELAY.error)OTU(DFSeriesBasic.SETENCODERDELAY.cmd.send)OTU(DFSeriesBasic.priv.busy)OTU(Domino_internal_setencoderdelay.ER);
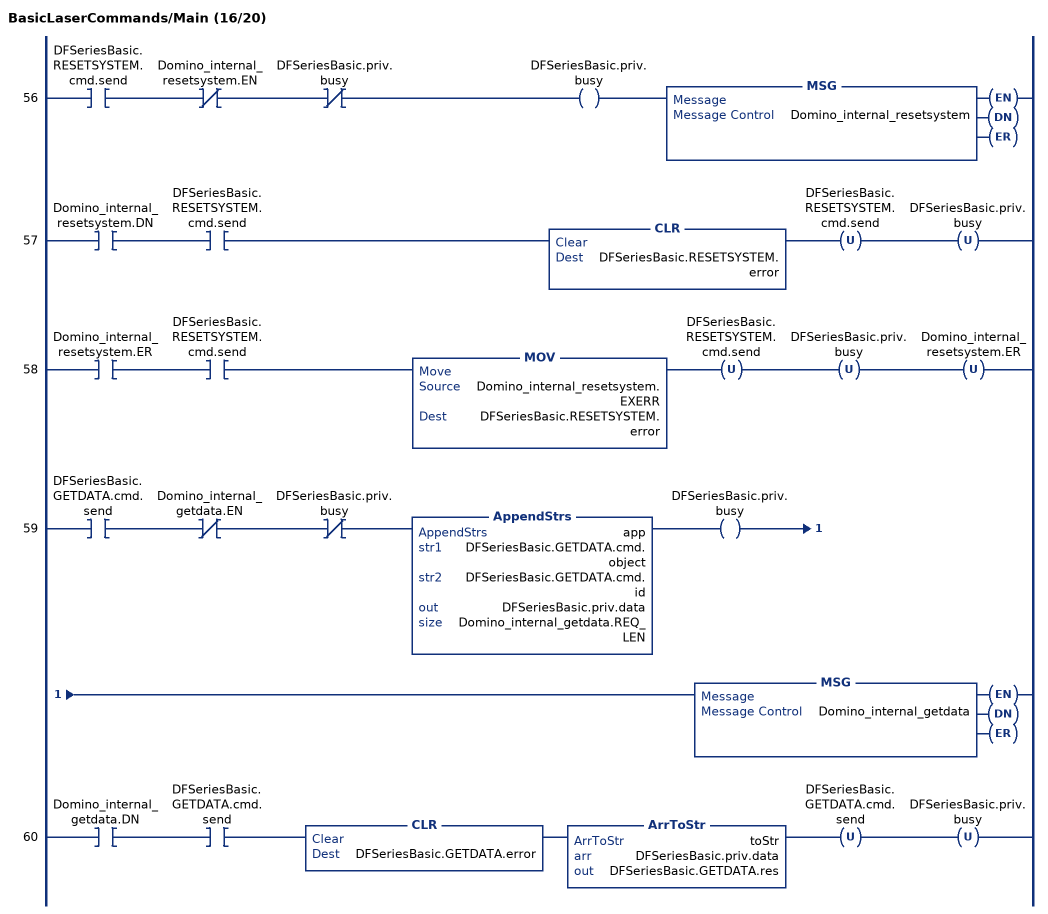
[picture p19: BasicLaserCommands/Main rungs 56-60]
   56: XIC(DFSeriesBasic.RESETSYSTEM.cmd.send)XIO(Domino_internal_resetsystem.EN)XIO(DFSeriesBasic.priv.busy)OTE(DFSeriesBasic.priv.busy)MSG(Domino_internal_resetsystem);
   57: XIC(Domino_internal_resetsystem.DN)XIC(DFSeriesBasic.RESETSYSTEM.cmd.send)CLR(DFSeriesBasic.RESETSYSTEM.error)OTU(DFSeriesBasic.RESETSYSTEM.cmd.send)OTU(DFSeriesBasic.priv.busy);
   58: XIC(Domino_internal_resetsystem.ER)XIC(DFSeriesBasic.RESETSYSTEM.cmd.send)MOV(Domino_internal_resetsystem.EXERR,DFSeriesBasic.RESETSYSTEM.error)OTU(DFSeriesBasic.RESETSYSTEM.cmd.send)OTU(DFSeriesBasic.priv.busy)OTU(Domino_internal_resetsystem.ER);
   59: XIC(DFSeriesBasic.GETDATA.cmd.send)XIO(Domino_internal_getdata.EN)XIO(DFSeriesBasic.priv.busy)AppendStrs(app,DFSeriesBasic.GETDATA.cmd.object,DFSeriesBasic.GETDATA.cmd.id,DFSeriesBasic.priv.data,Domino_internal_getdata.REQ_LEN)OTE(DFSeriesBasic.priv.busy)MSG(Domino_internal_getdata);
   60: XIC(Domino_internal_getdata.DN)XIC(DFSeriesBasic.GETDATA.cmd.send)CLR(DFSeriesBasic.GETDATA.error)ArrToStr(toStr,DFSeriesBasic.priv.data,DFSeriesBasic.GETDATA.res)OTU(DFSeriesBasic.GETDATA.cmd.send)OTU(DFSeriesBasic.priv.busy);
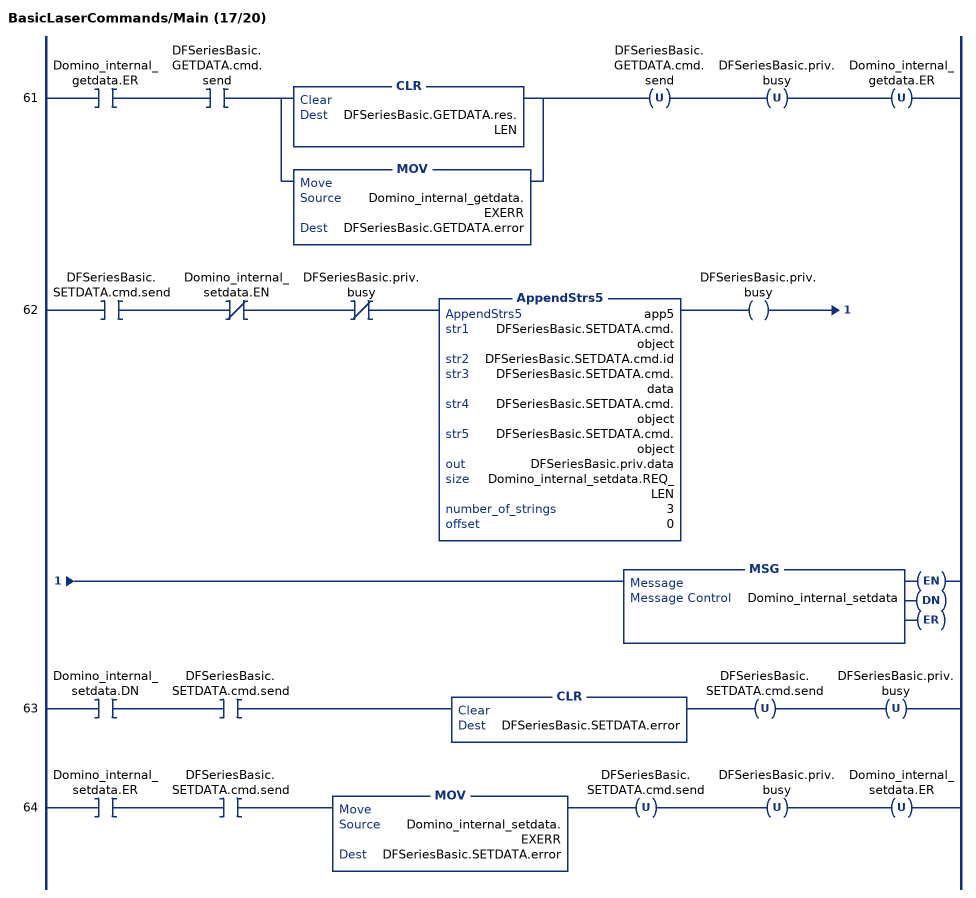
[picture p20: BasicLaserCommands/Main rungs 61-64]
   61: XIC(Domino_internal_getdata.ER)XIC(DFSeriesBasic.GETDATA.cmd.send)[CLR(DFSeriesBasic.GETDATA.res.LEN) ,MOV(Domino_internal_getdata.EXERR,DFSeriesBasic.GETDATA.error) ]OTU(DFSeriesBasic.GETDATA.cmd.send)OTU(DFSeriesBasic.priv.busy)OTU(Domino_internal_getdata.ER);
   62: XIC(DFSeriesBasic.SETDATA.cmd.send)XIO(Domino_internal_setdata.EN)XIO(DFSeriesBasic.priv.busy)AppendStrs5(app5,DFSeriesBasic.SETDATA.cmd.object,DFSeriesBasic.SETDATA.cmd.id,DFSeriesBasic.SETDATA.cmd.data,DFSeriesBasic.SETDATA.cmd.object,DFSeriesBasic.SETDATA.cmd.object,DFSeriesBasic.priv.data,Domino_internal_setdata.REQ_LEN,3,0)OTE(DFSeriesBasic.priv.busy)MSG(Domino_internal_setdata);
   63: XIC(Domino_internal_setdata.DN)XIC(DFSeriesBasic.SETDATA.cmd.send)CLR(DFSeriesBasic.SETDATA.error)OTU(DFSeriesBasic.SETDATA.cmd.send)OTU(DFSeriesBasic.priv.busy);
   64: XIC(Domino_internal_setdata.ER)XIC(DFSeriesBasic.SETDATA.cmd.send)MOV(Domino_internal_setdata.EXERR,DFSeriesBasic.SETDATA.error)OTU(DFSeriesBasic.SETDATA.cmd.send)OTU(DFSeriesBasic.priv.busy)OTU(Domino_internal_setdata.ER);
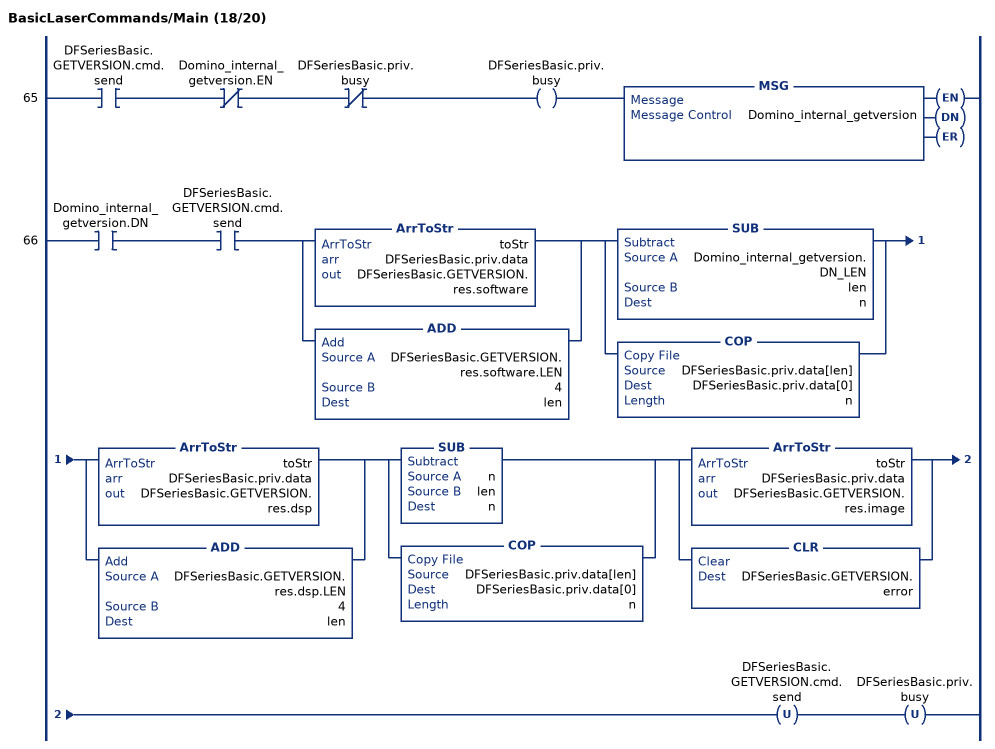
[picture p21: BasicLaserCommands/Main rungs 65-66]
   65: XIC(DFSeriesBasic.GETVERSION.cmd.send)XIO(Domino_internal_getversion.EN)XIO(DFSeriesBasic.priv.busy)OTE(DFSeriesBasic.priv.busy)MSG(Domino_internal_getversion);
   66: XIC(Domino_internal_getversion.DN)XIC(DFSeriesBasic.GETVERSION.cmd.send)[ArrToStr(toStr,DFSeriesBasic.priv.data,DFSeriesBasic.GETVERSION.res.software) ,ADD(DFSeriesBasic.GETVERSION.res.software.LEN,4,len) ][SUB(Domino_internal_getversion.DN_LEN,len,n) ,COP(DFSeriesBasic.priv.data[len],DFSeriesBasic.priv.data[0],n) ][ArrToStr(toStr,DFSeriesBasic.priv.data,DFSeriesBasic.GETVERSION.res.dsp) ,ADD(DFSeriesBasic.GETVERSION.res.dsp.LEN,4,len) ][SUB(n,len,n) ,COP(DFSeriesBasic.priv.data[len],DFSeriesBasic.priv.data[0],n) ][ArrToStr(toStr,DFSeriesBasic.priv.data,DFSeriesBasic.GETVERSION.res.image) ,CLR(DFSeriesBasic.GETVERSION.error) ]OTU(DFSeriesBasic.GETVERSION.cmd.send)OTU(DFSeriesBasic.priv.busy);
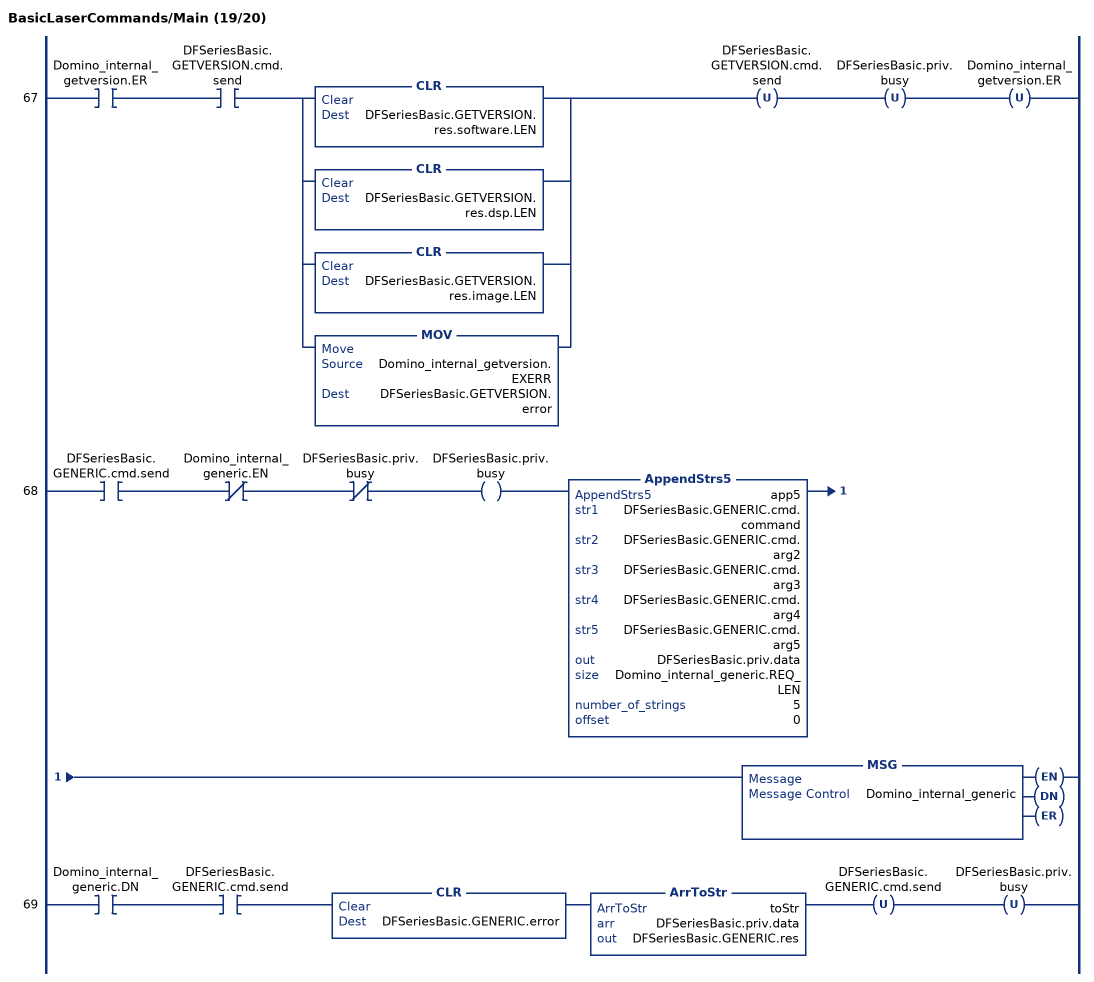
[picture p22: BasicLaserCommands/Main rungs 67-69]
   67: XIC(Domino_internal_getversion.ER)XIC(DFSeriesBasic.GETVERSION.cmd.send)[CLR(DFSeriesBasic.GETVERSION.res.software.LEN) ,CLR(DFSeriesBasic.GETVERSION.res.dsp.LEN) ,CLR(DFSeriesBasic.GETVERSION.res.image.LEN) ,MOV(Domino_internal_getversion.EXERR,DFSeriesBasic.GETVERSION.error) ]OTU(DFSeriesBasic.GETVERSION.cmd.send)OTU(DFSeriesBasic.priv.busy)OTU(Domino_internal_getversion.ER);
   68: XIC(DFSeriesBasic.GENERIC.cmd.send)XIO(Domino_internal_generic.EN)XIO(DFSeriesBasic.priv.busy)OTE(DFSeriesBasic.priv.busy)AppendStrs5(app5,DFSeriesBasic.GENERIC.cmd.command,DFSeriesBasic.GENERIC.cmd.arg2,DFSeriesBasic.GENERIC.cmd.arg3,DFSeriesBasic.GENERIC.cmd.arg4,DFSeriesBasic.GENERIC.cmd.arg5,DFSeriesBasic.priv.data,Domino_internal_generic.REQ_LEN,5,0)MSG(Domino_internal_generic);
   69: XIC(Domino_internal_generic.DN)XIC(DFSeriesBasic.GENERIC.cmd.send)CLR(DFSeriesBasic.GENERIC.error)ArrToStr(toStr,DFSeriesBasic.priv.data,DFSeriesBasic.GENERIC.res)OTU(DFSeriesBasic.GENERIC.cmd.send)OTU(DFSeriesBasic.priv.busy);
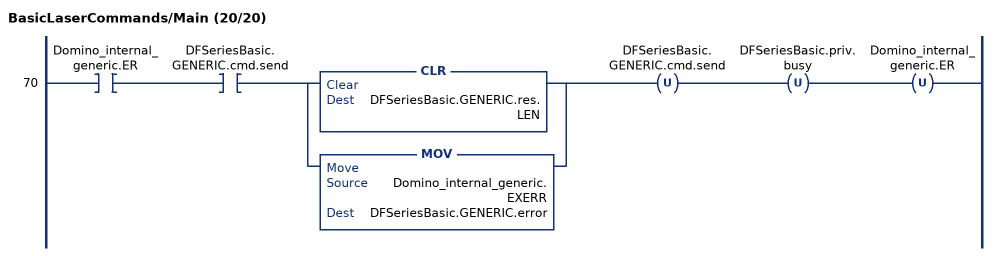
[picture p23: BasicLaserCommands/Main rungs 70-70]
   70: XIC(Domino_internal_generic.ER)XIC(DFSeriesBasic.GENERIC.cmd.send)[CLR(DFSeriesBasic.GENERIC.res.LEN) ,MOV(Domino_internal_generic.EXERR,DFSeriesBasic.GENERIC.error) ]OTU(DFSeriesBasic.GENERIC.cmd.send)OTU(DFSeriesBasic.priv.busy)OTU(Domino_internal_generic.ER);
END_ROUTINE
END_PROGRAM
